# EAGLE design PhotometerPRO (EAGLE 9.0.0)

## Sheet 1 of 6: Input - Relay
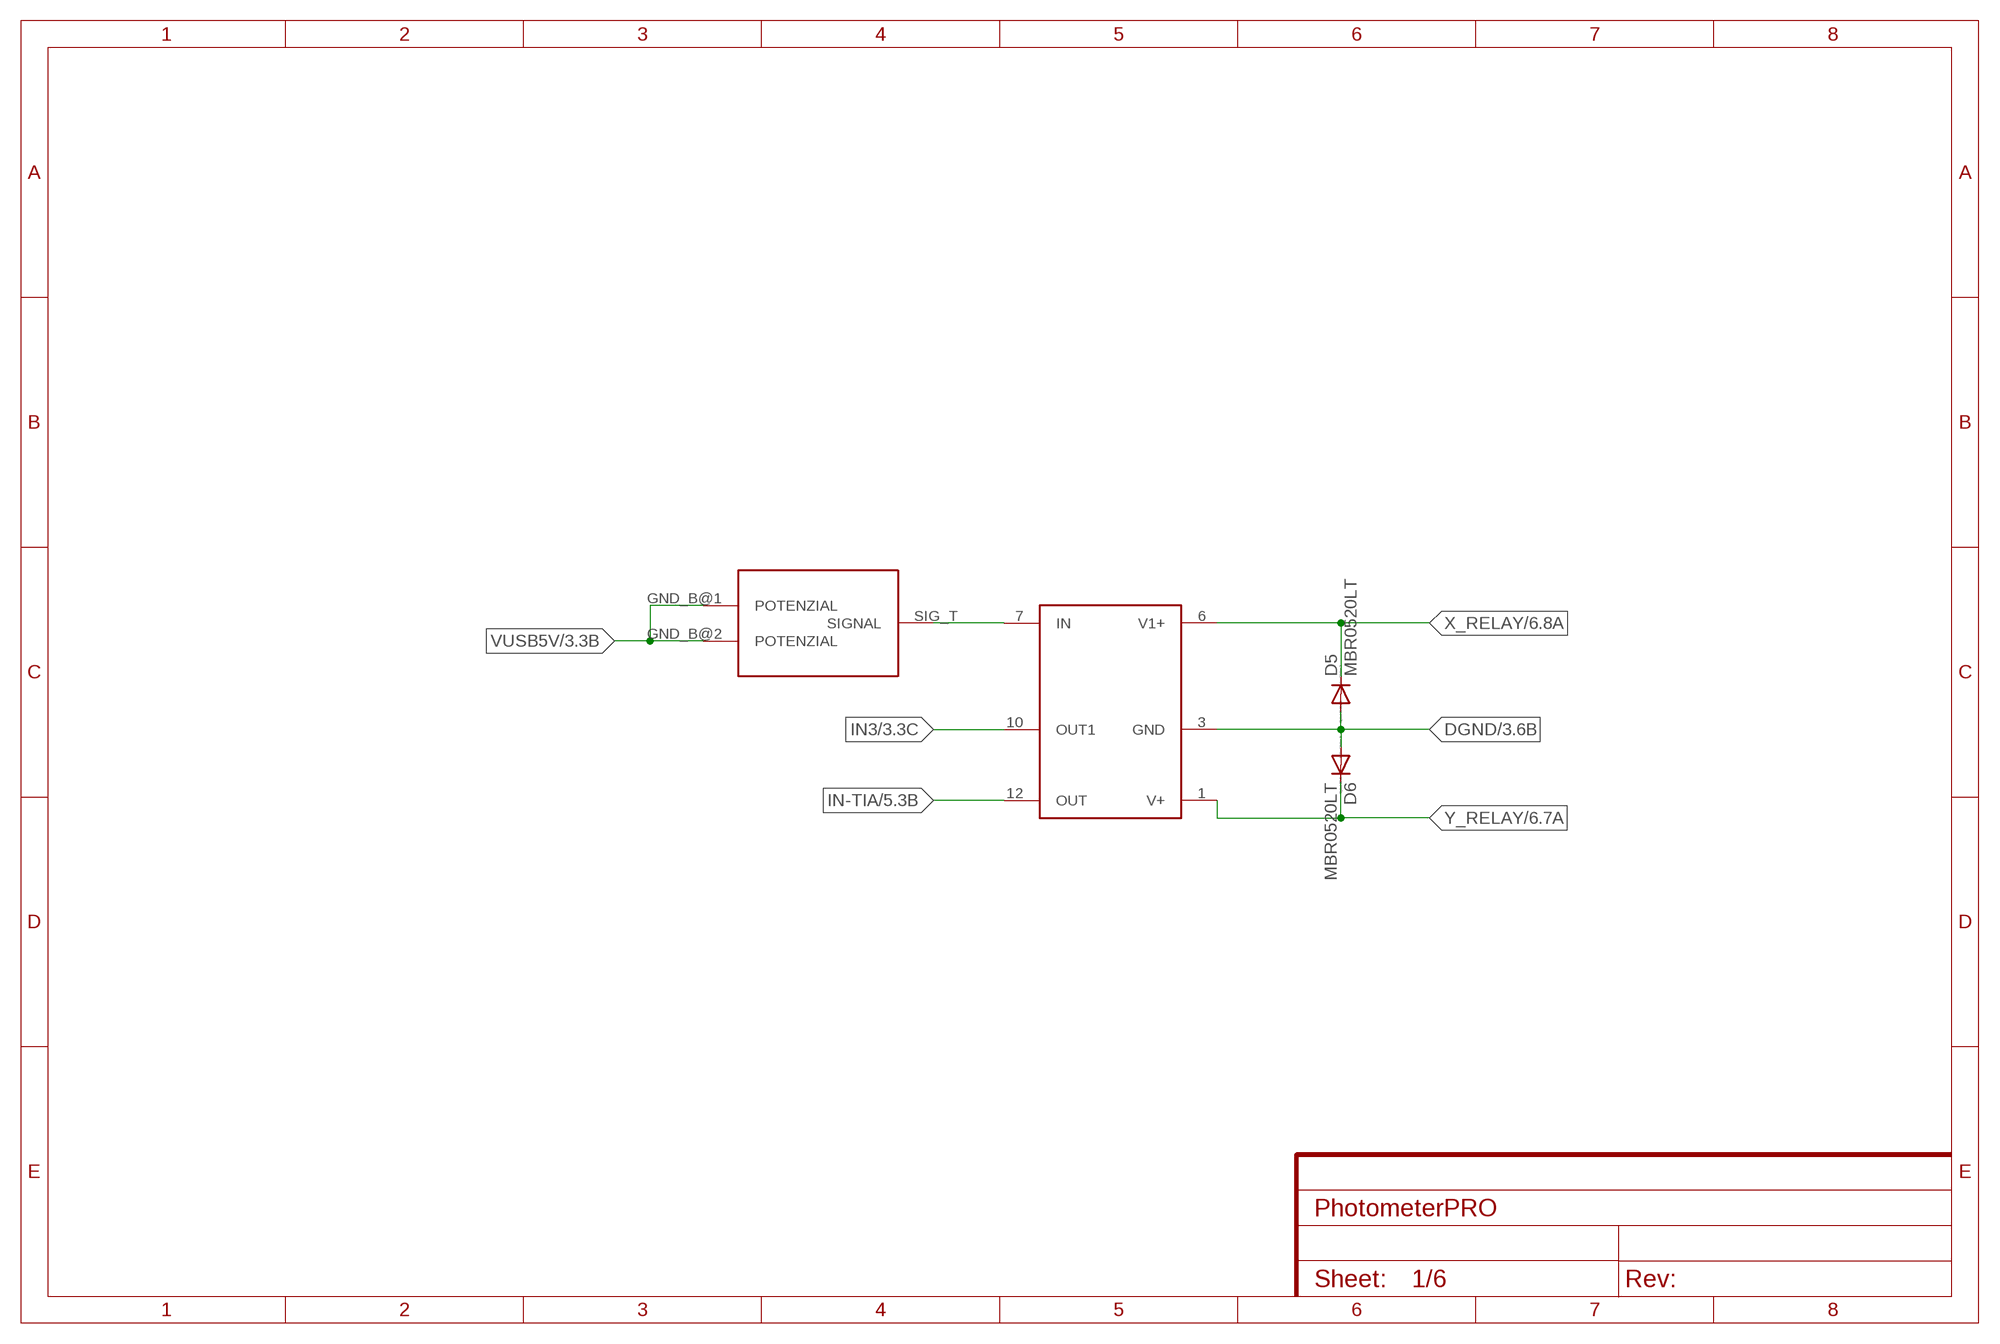
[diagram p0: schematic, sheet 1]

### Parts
CON  SMA_RAND  [SMA-RAND-PRINT]
D5  MBR0520LT  [SOD123]
D6  MBR0520LT  [SOD123]
RELAY  DS1E  [DIP12_8MM_X_13MM_DS1E]

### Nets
DGND: D5.A D6.A RELAY.3(GND) ; also sheet 3,4,6
IN3: RELAY.10(OUT1) ; also sheet 3
IN-TIA: RELAY.12(OUT) ; also sheet 5
IPD: CON.SIG_T(SIGNAL) RELAY.7(IN)
VUSB5V: CON.GND_B@1(POTENZIAL) CON.GND_B@2(POTENZIAL) ; also sheet 3,4,6
X_RELAY: D5.C RELAY.6(V1+) ; also sheet 6
Y_RELAY: D6.C RELAY.1(V+) ; also sheet 6

## Sheet 2 of 6: VFC
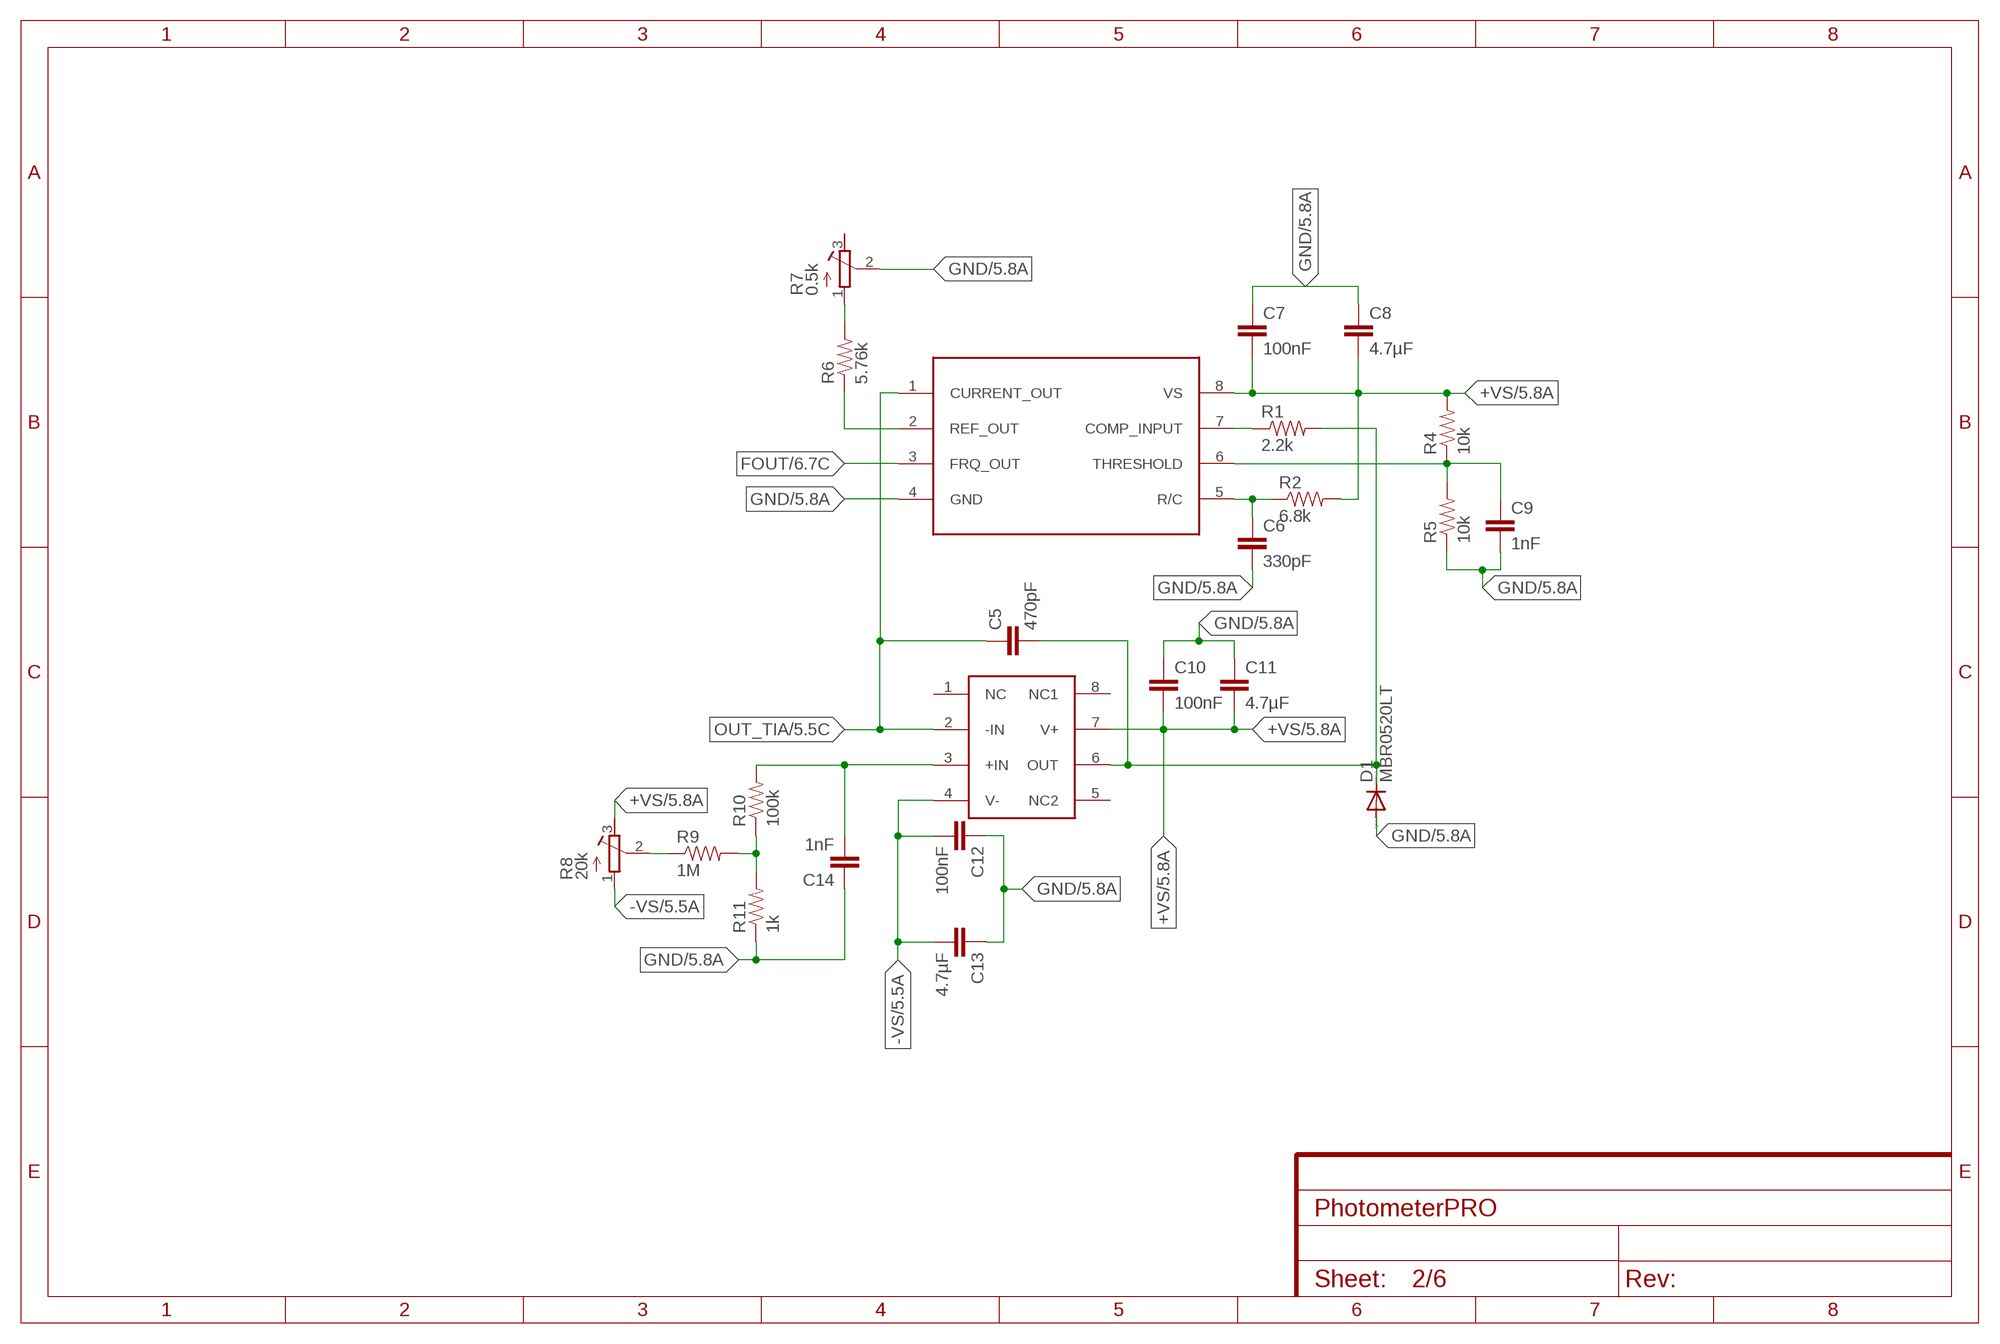
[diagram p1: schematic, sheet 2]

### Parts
C5  470pF  CAP0603-CAP  [0603-CAP]
C6  330pF  C-EUC0603K  [C0603K]
C7  100nF  C-EUC0603K  [C0603K]
C8  4.7µF  C-EUC0603K  [C0603K]
C9  1nF  C-EUC0603K  [C0603K]
C10  100nF  C-EUC0603K  [C0603K]
C11  4.7µF  C-EUC0603K  [C0603K]
C12  100nF  C-EUC0603K  [C0603K]
C13  4.7µF  C-EUC0603K  [C0603K]
C14  1nF  C-EUC0603K  [C0603K]
D1  MBR0520LT  [SOD123]
R1  2.2k  RESISTOR0603-RES  [0603-RES]
R2  6.8k  RESISTOR0805-RES  [0805]
R4  10k  RESISTOR0603-RES  [0603-RES]
R5  10k  RESISTOR0603-RES  [0603-RES]
R6  5.76k  RESISTOR0603-RES  [0603-RES]
R7  0.5k  R-TRIMMTSM53YL  [RTRIMTSM53YL]
R8  20k  R-TRIMMTS63Y  [RTRIMTS63Y]
R9  1M  RESISTOR0603-RES  [0603-RES]
R10  100k  RESISTOR0603-RES  [0603-RES]
R11  1k  RESISTOR0603-RES  [0603-RES]
U$10  OPA191  [SOIC8_4.90MMX3.91MM]
VFC  LM331  [DIP-08]

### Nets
+VS: C7.2 C8.2 C10.2 C11.2 R2.2 R4.2 R8.3(E) U$10.7(V+) VFC.8(VS) ; also sheet 5,6
-VS: C12.2 C13.2 R8.1(A) U$10.4(V-) ; also sheet 5,6
COMP_IN: R1.1 VFC.7(COMP_INPUT)
FOUT: VFC.3(FRQ_OUT) ; also sheet 6
GND: C6.2 C7.1 C8.1 C9.2 C10.1 C11.1 C12.1 C13.1 C14.1 D1.A R5.1 R7.2(S) R11.1 VFC.4(GND) ; also sheet 5,6
IN+INTE: C14.2 R10.2 U$10.3(+IN)
N$2: C5.2 D1.C R1.2 U$10.6(OUT)
N$8: C6.1 R2.1 VFC.5(R/C)
N$10: R6.1 VFC.2(REF_OUT)
N$11: C9.1 R4.1 R5.2 VFC.6(THRESHOLD)
N$12: R6.2 R7.1(A)
N$14: R9.2 R10.1 R11.2
N$15: R8.2(S) R9.1
OUT_TIA: C5.1 U$10.2(-IN) VFC.1(CURRENT_OUT) ; also sheet 5
Unconnected: R7.3(E) U$10.1(NC) U$10.5(NC2) U$10.8(NC1)

## Sheet 3 of 6: Mazet + Supply
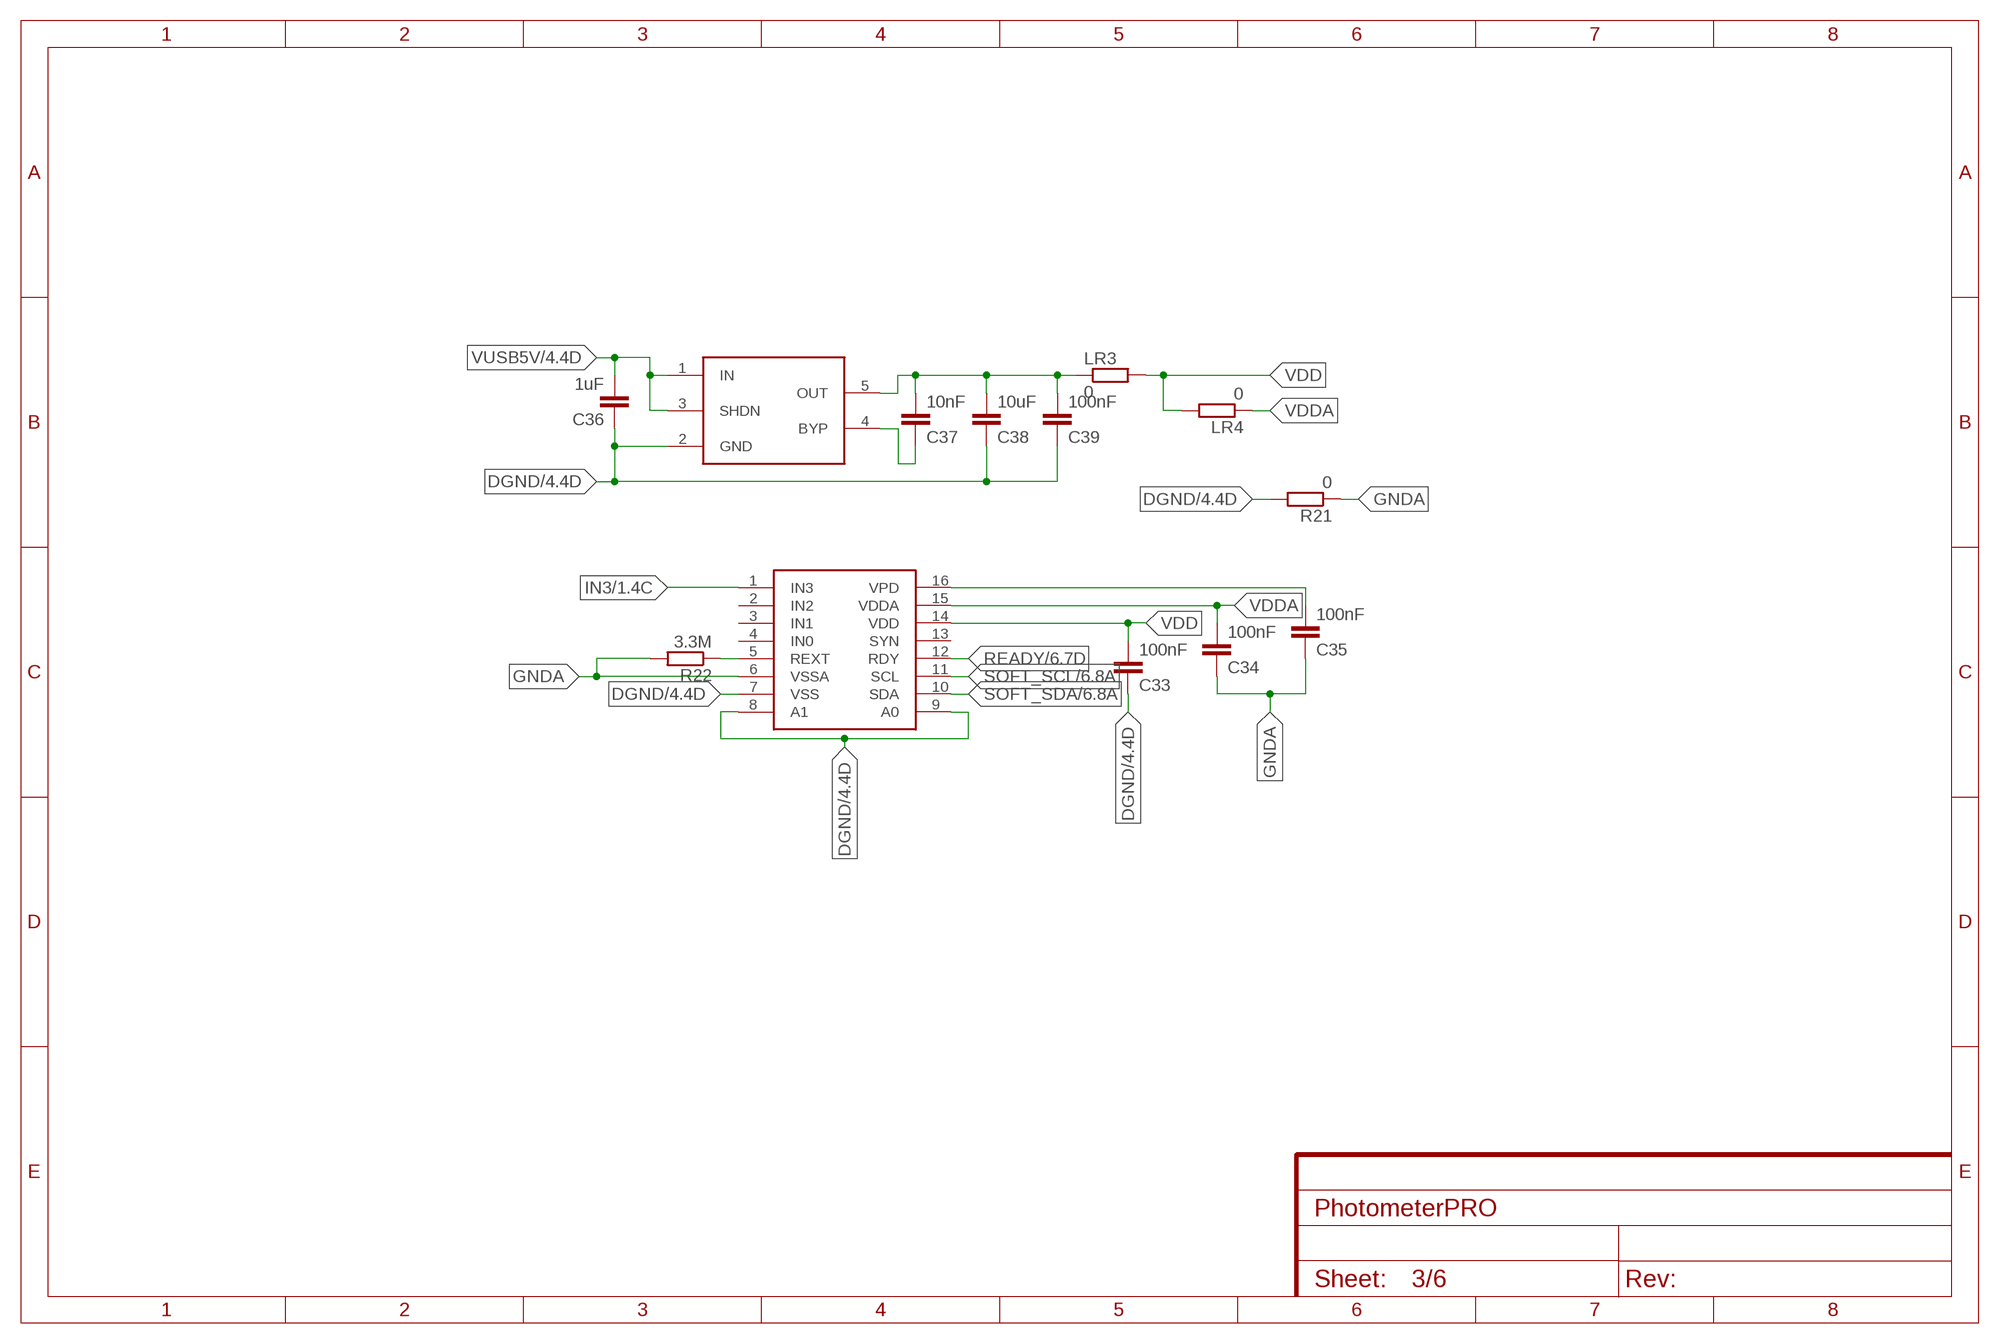
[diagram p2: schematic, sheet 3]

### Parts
C33  100nF  C-EUC0603  [C0603]
C34  100nF  C-EUC0603  [C0603]
C35  100nF  C-EUC0603  [C0603]
C36  1uF  C-EUC0603  [C0603]
C37  10nF  C-EUC0603  [C0603]
C38  10uF  C-EUC0603  [C0603]
C39  100nF  C-EUC0603  [C0603]
LDO1  LT1761  [TSOT23-5]
LR3  0  R-EU_R0603  [R0603]
LR4  0  R-EU_R0603  [R0603]
MCDC01  MCDC04  [SSOP16]
R21  0  R-EU_R0603  [R0603]
R22  3.3M  R-EU_R0603  [R0603]

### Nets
DGND: C33.1 C36.1 C38.1 C39.1 LDO1.2(GND) MCDC01.7(VSS) MCDC01.8(A1) MCDC01.9(A0) R21.2 ; also sheet 1,4,6
GNDA: C34.1 C35.1 MCDC01.6(VSSA) R21.1 R22.2
IN3: MCDC01.1(IN3) ; also sheet 1
LDO_OUT3V1: C37.2 C38.2 C39.2 LDO1.5(OUT) LR3.1
N$1: C37.1 LDO1.4(BYP)
READY: MCDC01.12(RDY) ; also sheet 6
REXT: MCDC01.5(REXT) R22.1
SOFT_SCL: MCDC01.11(SCL) ; also sheet 6
SOFT_SDA: MCDC01.10(SDA) ; also sheet 6
VDD: C33.2 LR3.2 LR4.2 MCDC01.14(VDD)
VDDA: C34.2 LR4.1 MCDC01.15(VDDA)
VPD: C35.2 MCDC01.16(VPD)
VUSB5V: C36.2 LDO1.1(IN) LDO1.3(SHDN) ; also sheet 1,4,6
Unconnected: MCDC01.2(IN2) MCDC01.3(IN1) MCDC01.4(IN0) MCDC01.13(SYN)

## Sheet 4 of 6: Display Joystik
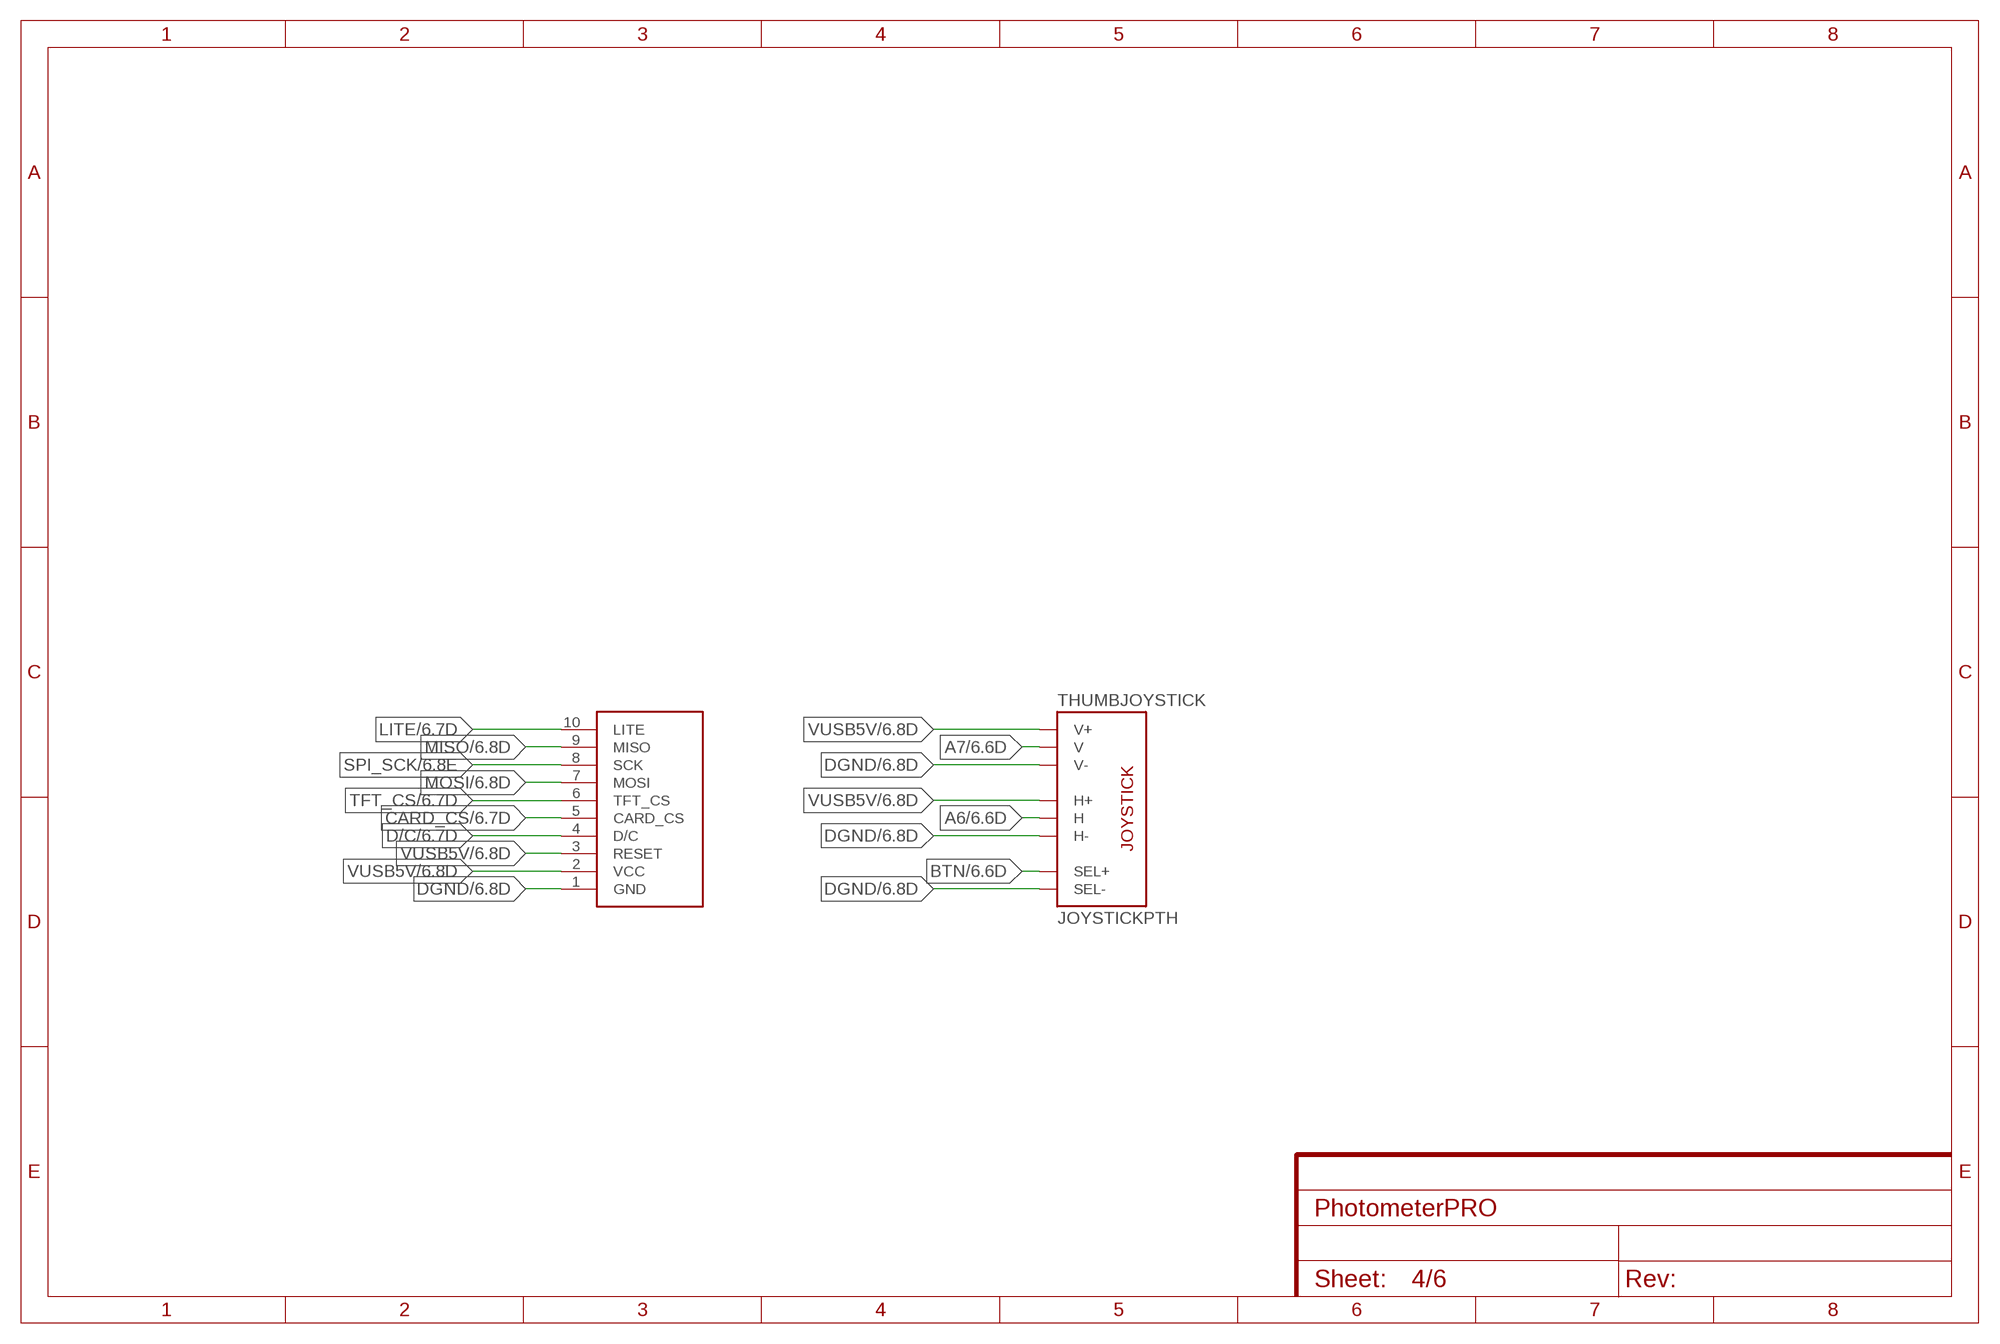
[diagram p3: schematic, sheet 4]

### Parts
DISPLAY  DISPLAY  [DISPLAY]
THUMBJOYSTICK  JOYSTICKPTH  [JOYSTICK]

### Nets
A6: THUMBJOYSTICK.H2(H) ; also sheet 6
A7: THUMBJOYSTICK.V2(V) ; also sheet 6
BTN: THUMBJOYSTICK.B1A(SEL+) ; also sheet 6
CARD_CS: DISPLAY.5(CARD_CS) ; also sheet 6
D/C: DISPLAY.4(D/C) ; also sheet 6
DGND: DISPLAY.1(GND) THUMBJOYSTICK.B2A(SEL-) THUMBJOYSTICK.H3(H-) THUMBJOYSTICK.V3(V-) ; also sheet 1,3,6
LITE: DISPLAY.10(LITE) ; also sheet 6
MISO: DISPLAY.9(MISO) ; also sheet 6
MOSI: DISPLAY.7(MOSI) ; also sheet 6
SPI_SCK: DISPLAY.8(SCK) ; also sheet 6
TFT_CS: DISPLAY.6(TFT_CS) ; also sheet 6
VUSB5V: DISPLAY.2(VCC) DISPLAY.3(RESET) THUMBJOYSTICK.H1(H+) THUMBJOYSTICK.V1(V+) ; also sheet 1,3,6

## Sheet 5 of 6: TIA
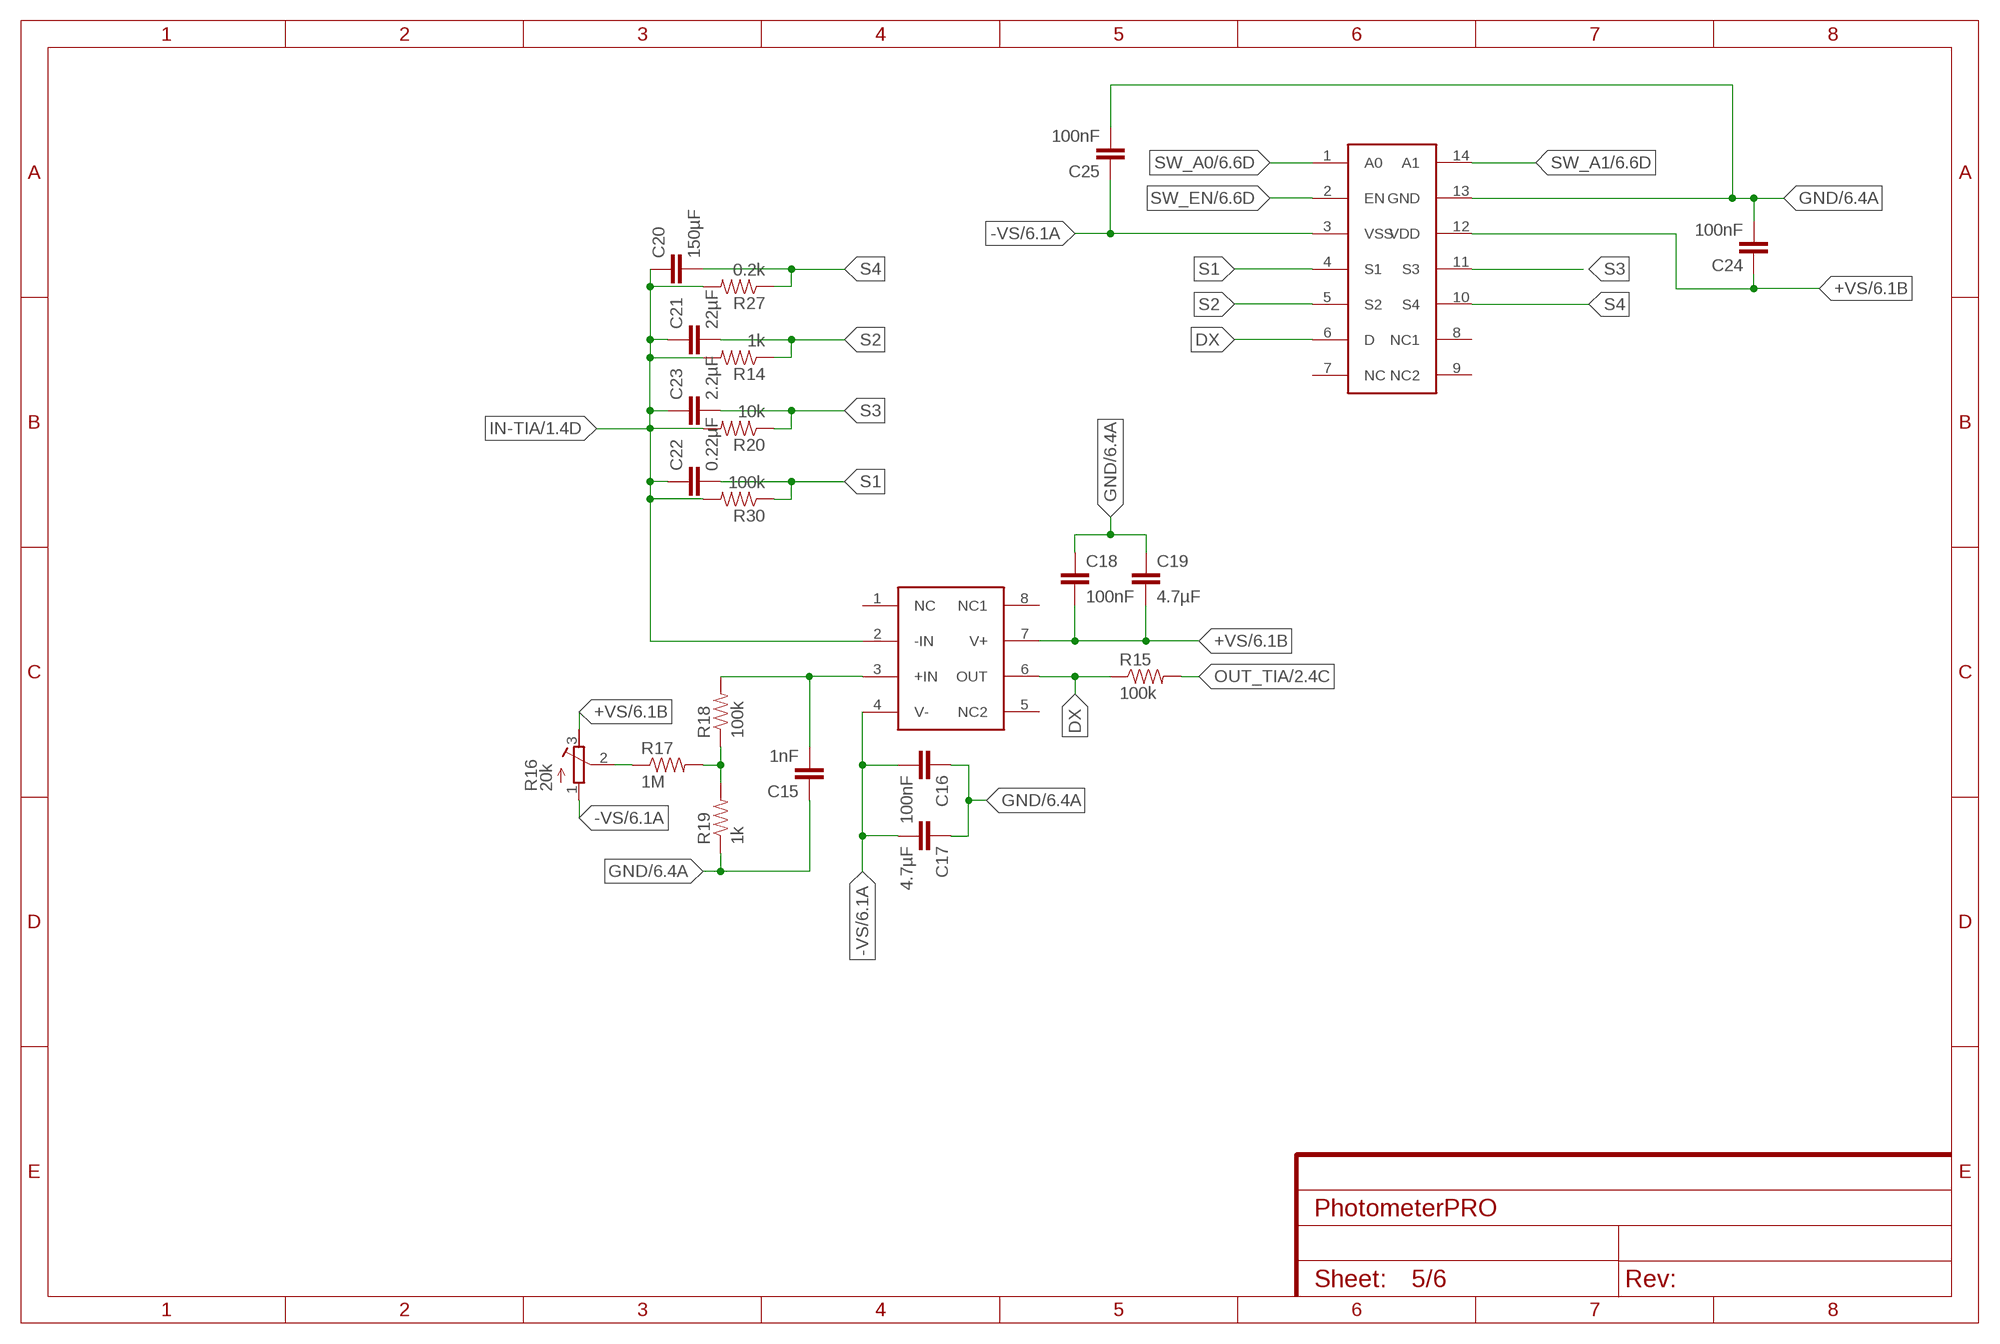
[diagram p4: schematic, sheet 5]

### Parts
C15  1nF  C-EUC0603K  [C0603K]
C16  100nF  C-EUC0603K  [C0603K]
C17  4.7µF  C-EUC0603K  [C0603K]
C18  100nF  C-EUC0603K  [C0603K]
C19  4.7µF  C-EUC0603K  [C0603K]
C20  150µF  C-EUC1206  [C1206]
C21  22µF  C-EUC0805  [C0805]
C22  0.22µF  C-EUC0603  [C0603]
C23  2.2µF  C-EUC0805  [C0805]
C24  100nF  C-EUC0603K  [C0603K]
C25  100nF  C-EUC0603K  [C0603K]
R14  1k  RESISTOR0603-RES  [0603-RES]
R15  100k  RESISTOR0603-RES  [0603-RES]
R16  20k  R-TRIMMTS63Y  [RTRIMTS63Y]
R17  1M  RESISTOR0603-RES  [0603-RES]
R18  100k  RESISTOR0603-RES  [0603-RES]
R19  1k  RESISTOR0603-RES  [0603-RES]
R20  10k  RESISTOR0603-RES  [0603-RES]
R27  0.2k  RESISTOR1206  [1206]
R30  100k  RESISTOR0603-RES  [0603-RES]
U$1  ADG1404  [TSSOP14-0.65-5X4.4MM]
U$12  OPA191  [SOIC8_4.90MMX3.91MM]

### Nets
+VS: C18.2 C19.2 C24.1 R16.3(E) U$1.12(VDD) U$12.7(V+) ; also sheet 2,6
-VS: C16.2 C17.2 C25.1 R16.1(A) U$1.3(VSS) U$12.4(V-) ; also sheet 2,6
DX: R15.1 U$1.6(D) U$12.6(OUT)
GND: C15.1 C16.1 C17.1 C18.1 C19.1 C24.2 C25.2 R19.1 U$1.13(GND) ; also sheet 2,6
IN+TIA: C15.2 R18.2 U$12.3(+IN)
IN-TIA: C20.1 C21.1 C22.1 C23.1 R14.2 R20.2 R27.2 R30.2 U$12.2(-IN) ; also sheet 1
N$21: R17.2 R18.1 R19.2
N$22: R16.2(S) R17.1
OUT_TIA: R15.2 ; also sheet 2
S1: C22.2 R30.1 U$1.4(S1)
S2: C21.2 R14.1 U$1.5(S2)
S3: C23.2 R20.1 U$1.11(S3)
S4: C20.2 R27.1 U$1.10(S4)
SW_A0: U$1.1(A0) ; also sheet 6
SW_A1: U$1.14(A1) ; also sheet 6
SW_EN: U$1.2(EN) ; also sheet 6
Unconnected: U$1.7(NC) U$1.8(NC1) U$1.9(NC2) U$12.1(NC) U$12.5(NC2) U$12.8(NC1)

## Sheet 6 of 6: µC-Nano Versorgung
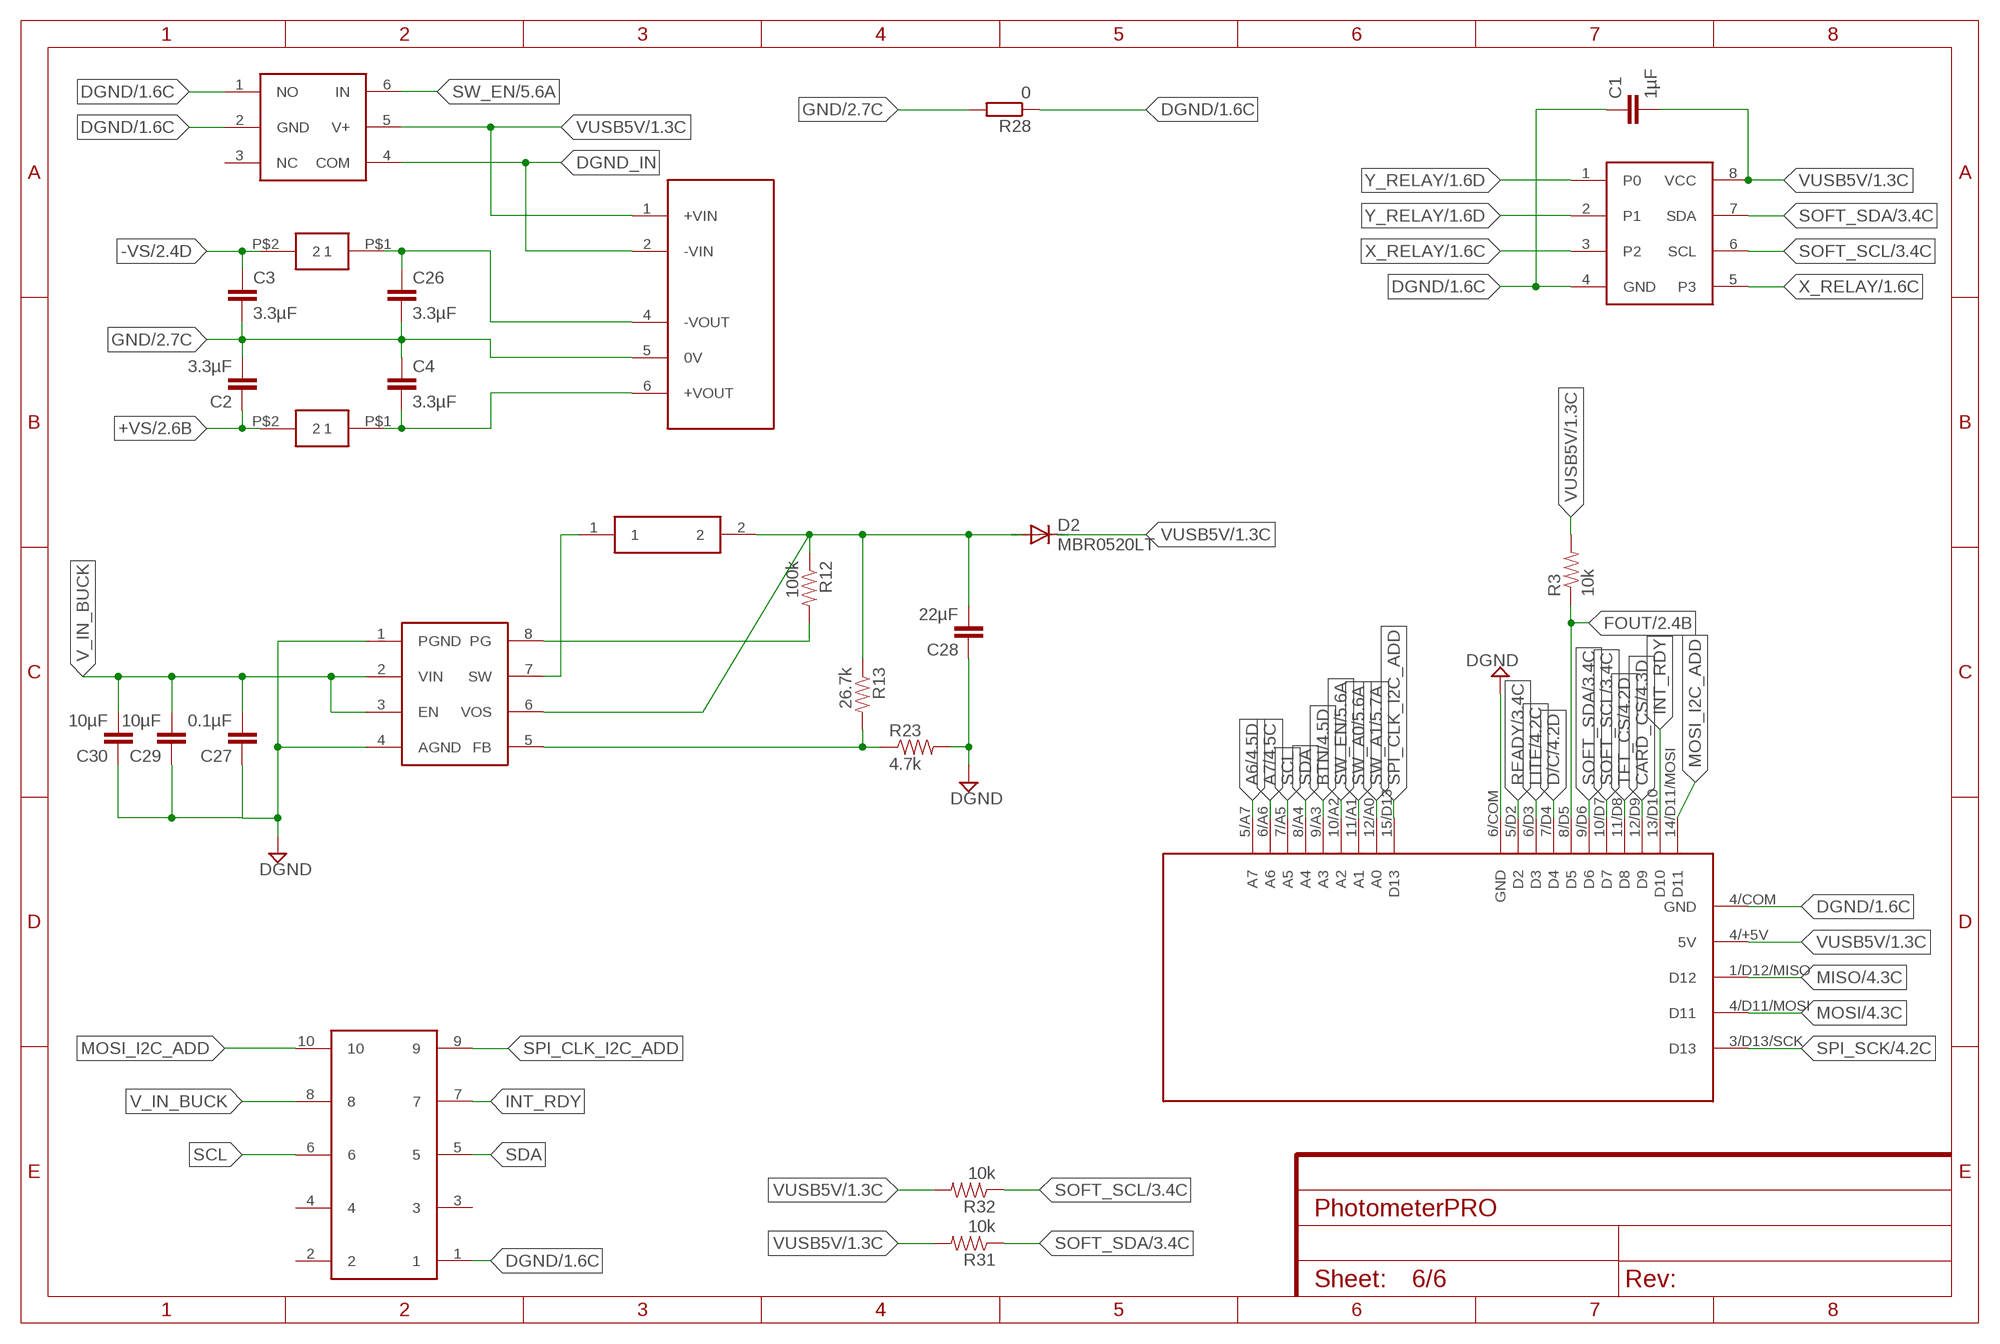
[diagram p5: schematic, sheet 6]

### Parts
C1  1µF  C-EUC0603K  [C0603K]
C2  3.3µF  C-EUC0603K  [C0603K]
C3  3.3µF  C-EUC0603K  [C0603K]
C4  3.3µF  C-EUC0603K  [C0603K]
C26  3.3µF  C-EUC0603K  [C0603K]
C27  0.1µF  C-EUC0603K  [C0603K]
C28  22µF  C-EUC0603K  [C0603K]
C29  10µF  C-EUC0603K  [C0603K]
C30  10µF  C-EUC0603K  [C0603K]
D2  MBR0520LT  [SOD123]
R3  10k  RESISTOR0603-RES  [0603-RES]
R12  100k  RESISTOR0603-RES  [0603-RES]
R13  26.7k  RESISTOR0603-RES  [0603-RES]
R23  4.7k  RESISTOR0603-RES  [0603-RES]
R28  0  R-EU_R0603  [R0603]
R31  10k  RESISTOR0603-RES  [0603-RES]
R32  10k  RESISTOR0603-RES  [0603-RES]
U$2  KMP_100µH  KMP  [KMP]
U$3  HEADER_10POL  [BOX_HEADER_2.54MM]
U$4  KMP_100µH  KMP  [KMP]
U$6  TS5A3159A  [SOT23-6]
U$7  0  PCA9536  [SOIC8_4.90MMX3.91MM]
U$9  LPS3015  [LPS3015]
U$11  NMA0515SC  [SIP7]
U$13  NANO_V2  [NANO_V2]
U$14  TPS62160  [POWER-SOP8]

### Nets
5.5VBUCK: C28.2 D2.A R12.1 R13.1 U$9.2 U$14.6(VOS)
+VS: C2.1 U$4.P$2 ; also sheet 2,5
-VS: C3.1 U$2.P$2 ; also sheet 2,5
A6: U$13.5/A7(A7) ; also sheet 4
A7: U$13.6/A6(A6) ; also sheet 4
BTN: U$13.9/A3(A3) ; also sheet 4
CARD_CS: U$13.12/D9(D9) ; also sheet 4
D/C: U$13.7/D4(D4) ; also sheet 4
DGND: C1.1 C27.1 C28.1 C29.1 C30.1 R23.2 R28.1 U$3.1 U$6.1(NO) U$6.2(GND) U$7.4(GND) U$13.4/COM(GND) U$13.6/COM(GND) U$14.1(PGND) U$14.4(AGND) ; also sheet 1,3,4
DGND_IN: U$6.4(COM) U$11.2(-VIN)
FOUT: R3.1 U$13.8/D5(D5) ; also sheet 2
GND: C2.2 C3.2 C4.1 C26.2 R28.2 U$11.5(0V) ; also sheet 2,5
INT_RDY: U$3.7 U$13.13/D10(D10)
LITE: U$13.6/D3(D3) ; also sheet 4
MISO: U$13.1/D12/MISO(D12) ; also sheet 4
MOSI: U$13.4/D11/MOSI(D11) ; also sheet 4
MOSI_I2C_ADD: U$3.10 U$13.14/D11/MOSI(D11)
N$4: C4.2 U$4.P$1 U$11.6(+VOUT)
N$6: C26.1 U$2.P$1 U$11.4(-VOUT)
N$7: R13.2 R23.1 U$14.5(FB)
N$17: R12.2 U$14.8(PG)
N$18: U$9.1 U$14.7(SW)
READY: U$13.5/D2(D2) ; also sheet 3
SCL: U$3.6 U$13.7/A5(A5)
SDA: U$3.5 U$13.8/A4(A4)
SOFT_SCL: R32.1 U$7.6(SCL) U$13.10/D7(D7) ; also sheet 3
SOFT_SDA: R31.1 U$7.7(SDA) U$13.9/D6(D6) ; also sheet 3
SPI_CLK_I2C_ADD: U$3.9 U$13.15/D13(D13)
SPI_SCK: U$13.3/D13/SCK(D13) ; also sheet 4
SW_A0: U$13.11/A1(A1) ; also sheet 5
SW_A1: U$13.12/A0(A0) ; also sheet 5
SW_EN: U$6.6(IN) U$13.10/A2(A2) ; also sheet 5
TFT_CS: U$13.11/D8(D8) ; also sheet 4
V_IN_BUCK: C27.2 C29.2 C30.2 U$3.8 U$14.2(VIN) U$14.3(EN)
VUSB5V: C1.2 D2.C R3.2 R31.2 R32.2 U$6.5(V+) U$7.8(VCC) U$11.1(+VIN) U$13.4/+5V(5V) ; also sheet 1,3,4
X_RELAY: U$7.3(P2) U$7.5(P3) ; also sheet 1
Y_RELAY: U$7.1(P0) U$7.2(P1) ; also sheet 1
Unconnected: U$3.2 U$3.3 U$3.4 U$6.3(NC)

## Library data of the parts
C1-C4 C6-C30 C33-C39 = rcl:C-EU: CAPACITOR, European symbol
C5 = SparkFun-Passives:CAP: Capacitor
CON = VFC_lib:SMA_RAND
D1 D2 D5 D6 = VFC_lib:MBR0520LT: SCHOTTKY BARRIER RECTIFIER
DISPLAY = Lego:DISPLAY
LDO1 = OpenPhotonicsLib:LT1761
LR3 LR4 R21 R22 = rcl:R-EU_: RESISTOR, European symbol
MCDC01 = BachelorLib:MCDC04
R1-R6 R9-R15 R17-R20 R23 R27 R30-R32 = SparkFun-Passives:RESISTOR: Resistor
R7 R8 R16 = resistor:R-TRIMM: Trimm resistor
R28 = resistor:R-EU_: RESISTOR, European symbol
RELAY = VFC_lib:DS1E
THUMBJOYSTICK = SparkFun-Electromechanical:JOYSTICK: Thumb Joystick Joystick commonly found in PS2 controllers. Two pots and a select switch. Footprint proven. Spark Fun Electronics SKU : COM-09032
U$1 = VFC_lib:ADG1404
U$2 U$4 = VFC_lib:KMP
U$3 = VFC_lib:HEADER_10POL
U$6 = VFC_lib:TS5A3159A
U$7 = VFC_lib:PCA9536
U$9 = VFC_lib:LPS3015
U$10 U$12 = VFC_lib:OPA191
U$11 = VFC_lib:NMA0515SC
U$13 = VFC_lib:NANO_V2
U$14 = VFC_lib:TPS62160
VFC = VFC_lib:LM331

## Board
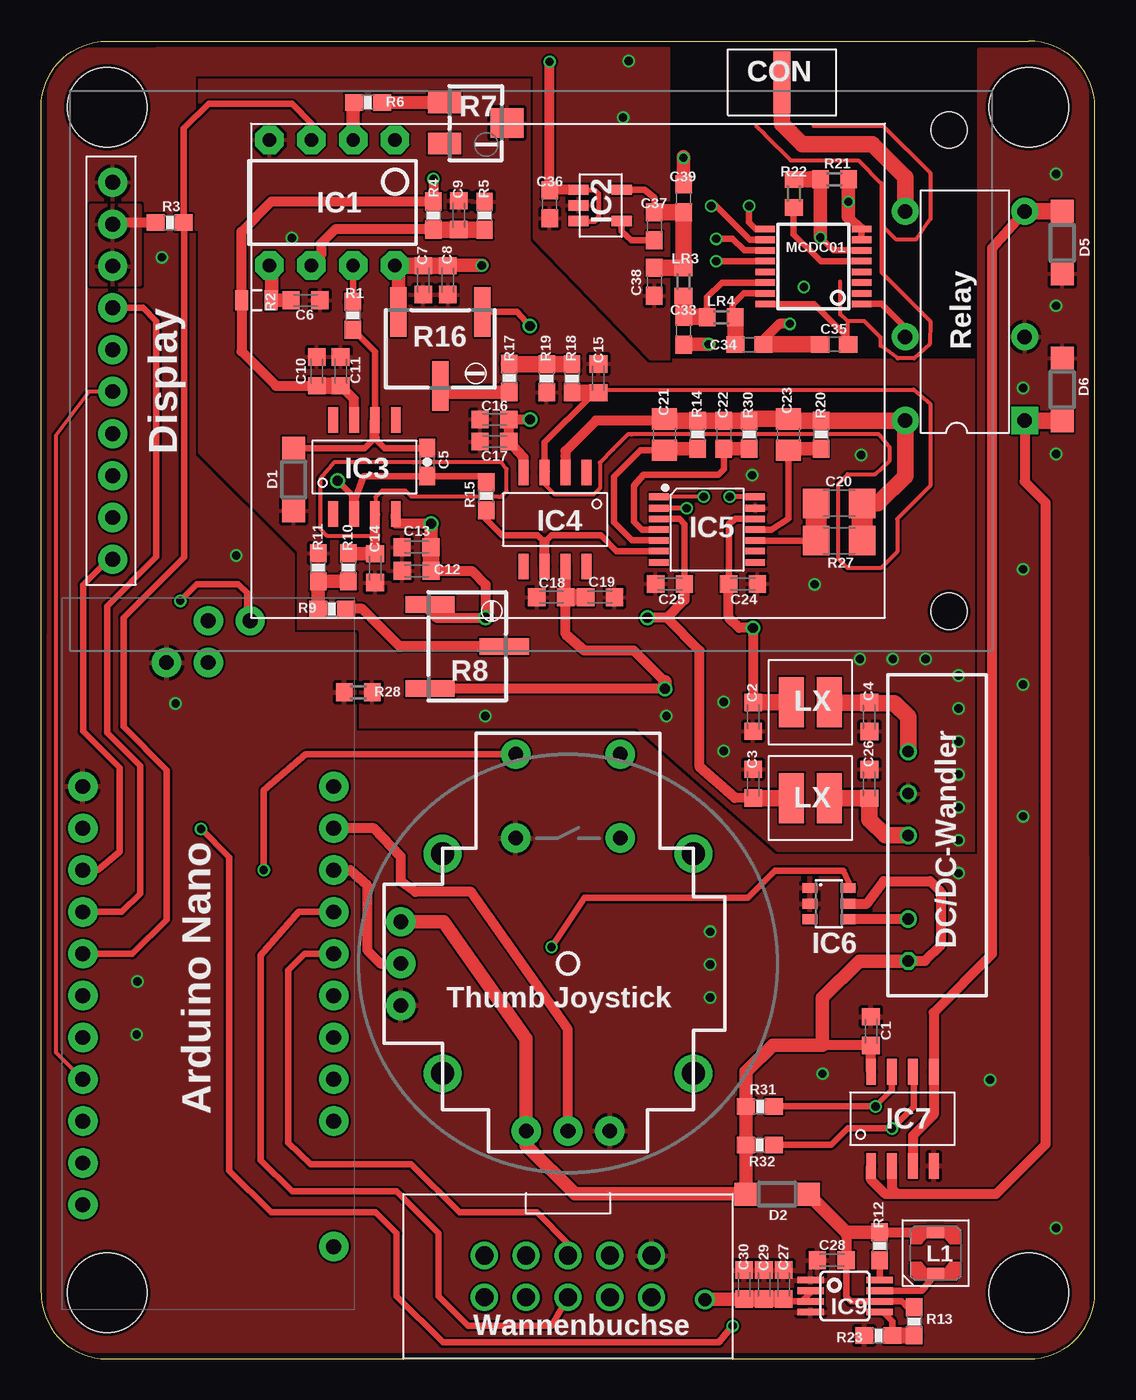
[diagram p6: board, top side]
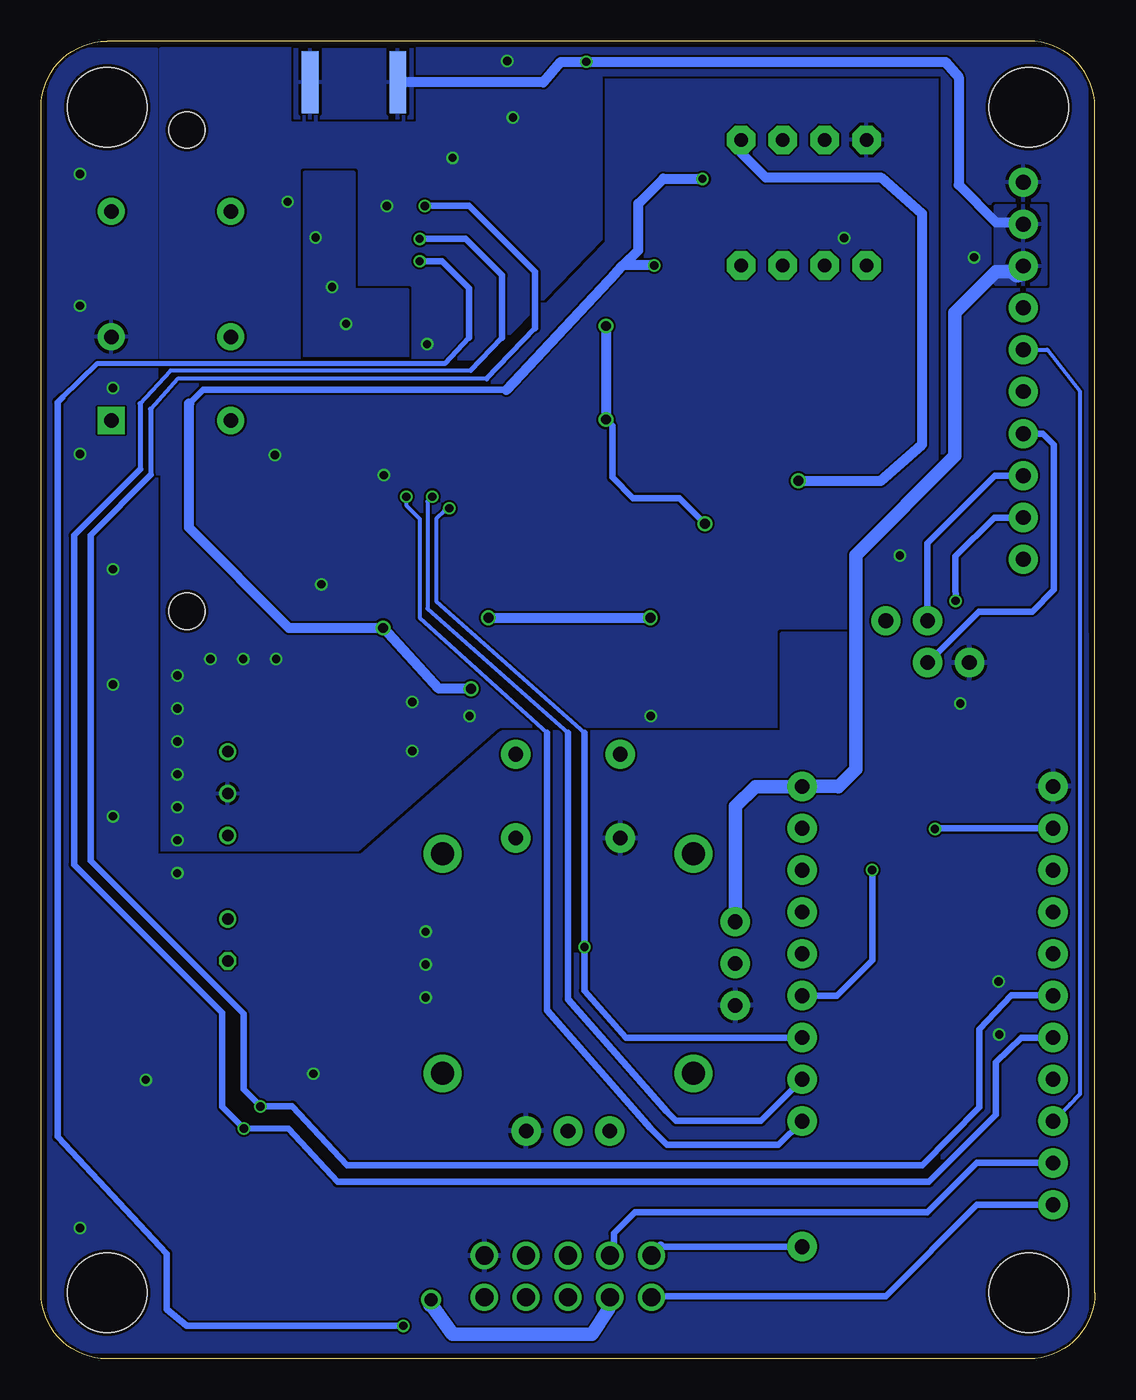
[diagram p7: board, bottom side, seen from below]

Size 64 x 80 mm. Coordinates in mm from the lower left corner, seen from the top.
Outline: 0,4 arc90 4,0 60,0 arc90 64,4 64,76 arc90 60,80 4,80 arc90 0,76 0,4
Copper layers (1*16): Top 0.018mm / dielectric 1.55mm / Bottom 0.018mm
Design rules "Multi-CB_2L_125um-Tracks_OL35um": minimum track width 0.125mm, minimum drill 0.2mm, track to track 0.125mm, track to pad 0.125mm, pad to pad 0.125mm, via to via 0.125mm, smd to smd 0mil, copper to edge 0.2mm, drill to drill 0.2mm, minimum pad ring 0.125mm, minimum via ring 0.125mm, stop-mask expansion 2mil, vias tented up to drill 0.45mm, thermal gap 0.2mm
Holes 4.82 mm at 4,76 60,76 60,4 4,4

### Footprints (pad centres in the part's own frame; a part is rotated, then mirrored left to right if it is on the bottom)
C0603K = smd 1.05 x 1.08: 1 -0.875,0; 2 0.875,0
0603-CAP = smd 1.1 x 1: 1 -0.85,0; 2 0.85,0
C1206 = smd 1.6 x 1.8: 1 -1.4,0; 2 1.4,0
C0805 = smd 1.3 x 1.5: 1 -0.95,0; 2 0.95,0
C0603 = smd 1.1 x 1: 1 -0.85,0; 2 0.85,0
SMA-RAND-PRINT = smd 3.75 x 1.02 bottom: GND_B@1 0,2.665; GND_B@2 0,-2.665 | smd 3.75 x 1.02: SIG_T 0,0
SOD123 = smd 1.4 x 1.4: A 1.9,0; C -1.9,0
DISPLAY = drill 0.9 pad 1.778: 1 -25.4,11.43; 2 -25.4,8.89; 3 -25.4,6.35; 4 -25.4,3.81; 5 -25.4,1.27; 6 -25.4,-1.27; 7 -25.4,-3.84; 8 -25.4,-6.38; 9 -25.4,-8.92; 10 -25.4,-11.46 | hole 2.2: 25.4,-14.605; 25.4,14.605
TSOT23-5 = smd 0.62 x 1.22: 1 0,-2.62; 2 0.95,-2.62; 3 1.9,-2.62; 4 1.9,0; 5 0,0
R0603 = smd 1 x 1.1: 1 -0.85,0; 2 0.85,0
SSOP16 = smd 0.4 x 1.2: 1 -2.275,-2.925; 2 -1.625,-2.925; 3 -0.975,-2.925; 4 -0.325,-2.925; 5 0.325,-2.925; 6 0.975,-2.925; 7 1.625,-2.925; 8 2.275,-2.925; 9 2.275,2.925; 10 1.625,2.925; 11 0.975,2.925; 12 0.325,2.925; 13 -0.325,2.925; 14 -0.975,2.925; 15 -1.625,2.925; 16 -2.275,2.925
0603-RES = smd 1.1 x 1: 1 -0.85,0; 2 0.85,0
0805 = smd 0.8 x 1.2: 1 -0.9,0; 2 0.9,0
RTRIMTSM53YL = smd 1.3 x 2: 1 -1.25,-1.9; 3 1.25,-1.9 | smd 1.8 x 2: 2 0,1.9
RTRIMTS63Y = smd 1 x 3: 1 -2.55,-2.25; 2 0,2.25; 3 2.55,-2.25
1206 = smd 1.6 x 1.8: 1 -1.4,0; 2 1.4,0
DIP12_8MM_X_13MM_DS1E = drill 0.889 pad 1.651 square: 1 -7.62,-4.128 | drill 0.889 pad 1.651: 3 -2.54,-4.128; 6 5.08,-4.128; 7 5.08,3.127; 10 -2.54,3.127; 12 -7.62,3.127
JOYSTICK = drill 0.9 pad 1.778: B1A -3.175,12.7; B1B 3.175,12.7; B2A -3.175,7.62; B2B 3.175,7.62 | drill 0.889 pad 1.778: H1 -2.54,-10.16; H2 0,-10.16; H3 2.54,-10.16; V1 -10.16,2.54; V2 -10.16,0; V3 -10.16,-2.54 | drill 1.397 pad 2.286: MOUNT1 -7.62,6.668; MOUNT2 -7.62,-6.668; MOUNT3 7.62,-6.668; MOUNT4 7.62,6.668
TSSOP14-0.65-5X4.4MM = smd 0.4 x 1.2: 1 -2,-2.925; 2 -1.3,-2.925; 3 -0.65,-2.925; 4 0,-2.925; 5 0.65,-2.925; 6 1.3,-2.925; 7 2,-2.925; 8 2,2.925; 9 1.3,2.925; 10 0.65,2.925; 11 0,2.925; 12 -0.65,2.925; 13 -1.3,2.925; 14 -2,2.925
KMP = smd 1.52 x 3.05: P$1 -1.145,0; P$2 1.145,0
BOX_HEADER_2.54MM = drill 1.1: 1 -1.27,5.08; 2 1.27,5.08; 3 -1.27,2.54; 4 1.27,2.54; 5 -1.27,0; 6 1.27,0; 7 -1.27,-2.54; 8 1.27,-2.54; 9 -1.27,-5.08; 10 1.27,-5.08
SOT23-6 = smd 0.6 x 0.9: 1 -0.95,-1.15; 2 0,-1.15; 3 0.95,-1.15; 4 0.95,1.15; 5 0,1.15; 6 -0.95,1.15
SOIC8_4.90MMX3.91MM = smd 0.6 x 1.55: 1 -1.27,-5.715; 2 0,-5.715; 3 1.27,-5.715; 4 2.54,-5.715; 5 2.54,0; 6 1.27,0; 7 0,0; 8 -1.27,0
LPS3015 = smd 0.76 x 1.02: 1 -1.27,0; 2 1.27,0.01
SIP7 = drill 0.7 pad 1.016 octagon: 1 -7.62,1.75 | drill 0.7 pad 1.016: 2 -5.08,1.75; 4 0,1.75; 5 2.54,1.75; 6 5.08,1.75
NANO_V2 = drill 0.9 pad 1.778: 1/D12/MISO 41.808,6.35; 3/D13/SCK 41.808,8.89; 4/+5V 31.75,1.27; 4/COM 31.75,16.51; 4/D11/MOSI 39.268,8.89; 5/A7 29.21,1.27; 5/D2 29.21,16.51; 6/A6 26.67,1.27; 6/COM 39.268,11.43; 6/D3 26.67,16.51; 7/A5 24.13,1.27; 7/D4 24.13,16.51; 8/A4 21.59,1.27; 8/D5 21.59,16.51; 9/A3 19.05,1.27; 9/D6 19.05,16.51; 10/A2 16.51,1.27; 10/D7 16.51,16.51; 11/A1 13.97,1.27; 11/D8 13.97,16.51; 12/A0 11.43,1.27; 12/D9 11.43,16.51; 13/D10 8.89,16.51; 14/D11/MOSI 6.35,16.51; 15/D13 3.81,1.27
POWER-SOP8 = smd 0.4 x 1.6: 1 -0.975,-2.1; 2 -0.325,-2.1; 3 0.325,-2.1; 4 0.975,-2.1; 5 0.975,2.1; 6 0.325,2.1; 7 -0.325,2.1; 8 -0.975,2.1
DIP-08 = drill 0.813 pad 1.727 octagon: 1 -3.81,-3.81; 2 -1.27,-3.81; 3 1.27,-3.81; 4 3.81,-3.81; 5 3.81,3.81; 6 1.27,3.81; 7 -1.27,3.81; 8 -3.81,3.81

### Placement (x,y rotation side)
C1  50.41,19.9 270 top
C2  43.24,38.98 270 top
C3  43.24,34.92 90 top
C4  50.3,38.97 90 top
C5  23.44,54.45 90 top
C6  16.05,64.26 0 top
C7  23.21,65.49 90 top
C8  24.7,65.49 90 top
C9  25.37,69.43 90 top
C10  16.74,59.95 270 top
C11  18.19,59.95 270 top
C12  22.81,47.84 0 top
C13  22.8,49.28 0 top
C14  20.29,48.01 90 top
C15  33.85,59.53 270 top
C16  27.53,57.03 0 top
C17  27.53,55.69 0 top
C18  30.98,46.24 0 top
C19  33.95,46.25 180 top
C20  48.47,51.94 180 top
C21  37.86,56.11 270 top
C22  41.47,56.11 270 top
C23  45.38,56.11 270 top
C24  42.63,47.04 0 top
C25  38.2,47.04 180 top
C26  50.3,34.91 90 top
C27  45.09,4.52 270 top
C28  48.03,5.98 0 top
C29  43.9,4.51 270 top
C30  42.7,4.51 270 top
C33  39.01,62.41 90 top
C34  43.02,61.58 180 top
C35  48.17,61.58 0 top
C36  30.88,70.11 90 top
C37  37.25,68.76 90 top
C38  37.25,65.39 90 top
C39  39.01,70.46 270 top
CON  45,77.5 90 top
D1  15.34,53.39 270 top
D2  44.71,10 0 top
D5  62.01,67.77 270 top
D6  62.01,58.85 90 top
DISPLAY  29.75,60 0 top
LDO1  35.26,70.98 270 top
LR3  39.01,65.39 270 top
LR4  41.31,63.24 180 top
MCDC01  46.91,66.32 90 top
R1  18.94,63.34 270 top
R2  13.08,64.26 180 top
R3  7.81,68.99 180 top
R4  23.83,69.42 90 top
R5  26.93,69.41 270 top
R6  19.85,76.28 0 top
R7  26.39,75.03 270 top
R8  25.87,43.26 270 top
R9  17.66,45.53 180 top
R10  18.67,48.06 90 top
R11  16.82,48.05 270 top
R12  50.93,6.85 270 top
R13  53.02,2.27 270 top
R14  39.87,56.11 90 top
R15  27.03,52.38 90 top
R16  24.25,61.31 180 top
R17  28.45,59.55 90 top
R18  32.24,59.53 270 top
R19  30.7,59.53 90 top
R20  47.37,56.11 90 top
R21  48.18,71.62 0 top
R22  45.72,70.75 90 top
R23  50.86,1.4 180 top
R27  48.47,49.68 0 top
R28  19.26,40.47 0 top
R30  43.02,56.11 90 top
R31  43.66,15.32 180 top
R32  43.65,12.98 180 top
RELAY  55.61,64.59 90 top
THUMBJOYSTICK  32,24 0 top
U$1  40.45,50.34 270 top
U$2  46.72,34.04 180 top
U$3  32,5 270 top
U$4  46.72,39.86 180 top
U$6  47.85,27.64 270 top
U$7  51.68,17.43 0 top
U$9  54.33,6.42 90 top
U$10  19,57 0 top
U$11  54.42,31.78 90 top
U$12  31.85,48.1 180 top
U$13  19.04,3 90 top
U$14  48.83,3.81 270 top
VFC  17.68,70.2 180 top

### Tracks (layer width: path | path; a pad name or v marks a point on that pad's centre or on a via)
5.5VBUCK
  Top 0.406: C28.2 48.9,3.76 49.17,3.48 U$14.6 52.27,3.48 52.64,3.11 R13.1
  Top 0.61: R12.1 52.97,7.7 U$9.2 | 49.06,7.7 48.9,7.49 C28.2
  Top 0.813: R12.1 49.06,7.7 48.92,7.7 D2.A | C28.2
  Top 1.016: 46.64,9.98 D2.A
+VS  (via drill 0.5, 0.6)
  Top 0.406: U$1.12 42.16,50.99 41.77,50.7 41.77,47.05 C24.1
  Top 0.61: U$4.P$2 45.58,40.31 | U$4.P$2 | U$4.P$2 | C24.1 41.76,45.03 42.41,44.38 v43.23,44.38 43.23,39.87 | v37.89,40.69 22.64,40.69 R8.3 | 14,70.27 12.18,68.43 R2.2 12.18,61.17 14.27,59.08 C10.2 16.75,59.06 | U$12.7 31.85,46.25 C18.2 | U$10.7 19,58.27 C11.2 | 37.89,41.11 36,43 33,43 31.85,44 31.85,46.1 C18.2 | C18.2 | v23.83,71.64 R4.2 23.85,70.27 23.85,70.28 14,70.28 14,70.27 | 14,70.27
  Top 0.813: 43.23,39.87 C2.1 | 24.69,66.36 C8.2 | C8.2 | v37.89,40.69 37.89,41.11 | v26.77,66.38 24.72,66.38 C8.2 | R16.3 21.71,66.17 VFC.8 | C10.2
  Top 1.016: C2.1 U$4.P$2 | C10.2 C11.2 | C19.2 C18.2 | 24.69,66.36 23.23,66.36 C7.2 21.51,66.37 VFC.8
  Bottom 0.406: 35.74,58.83 54.17,58.83 55,58
  Bottom 0.61: 35.74,58.83 29.1,65.94 | 29.1,65.94 29,66.04 | v37.89,40.69 39.86,40.69 v43.23,44.38 48.95,44.38 55.01,50.46 55.01,57.99 55,58 | 28.65,66.38 27.73,67.31 27.73,70.13 26.2,71.66 23.85,71.66 v23.83,71.64 | v26.77,66.38 28.65,66.38 | 28.65,66.38 29.1,65.94
-VS  (via drill 0.6)
  Top 0.406: U$1.3 38.76,50.99 39.08,50.68 C25.1 | R16.1 28.89,63.57 v29.68,62.71
  Top 0.61: 43.33,34.04 C3.1 42.14,34.06 39.99,35.94 40,43 38,45 | 22.62,45.81 R8.1 23.19,45.81 24,45 v27,45 27,47 26.16,47.84 C12.2 23.67,47.85 | C25.1 39.08,46.08 38,45 | 38,45 v36.84,45 | 21.56,51.3 U$10.4 21.54,50.71 v23.68,50.71 | 23.68,49.3 C13.2 | v29.69,57.03 C16.2 C17.2 29.31,54.71 U$12.4
  Top 0.813: v23.68,50.71 23.68,49.3
  Top 1.016: U$2.P$2 43.33,34.04 | C13.2 23.67,47.85
  Bottom 0.406: v23.68,50.71 25.24,52.26 28.05,52.26 29.31,53.52 29.31,56.64 v29.69,57.03
  Bottom 0.61: v36.84,45 v27,45 | v29.68,62.71 v29.69,57.03
A6
  Top 0.61: THUMBJOYSTICK.H2 32,20 26.12,28.35 22.74,28.35 21.84,29 21.84,30.5 20.23,32.21 U$13.5/A7
  Top 0.813: U$13.5/A7
A7
  Top 0.61: U$13.6/A6 18.77,29.67 19.8,28.74 19.8,24.81 20.61,24 THUMBJOYSTICK.V2
BTN  (via drill 0.5)
  Top 0.406: THUMBJOYSTICK.B1A 16.05,36.7 13.52,34.52 v13.52,29.68
  Bottom 0.254: THUMBJOYSTICK.B1A 28.82,36.83
  Bottom 0.406: v13.52,29.68 13.52,24.19 15.65,22.05 U$13.9/A3
CARD_CS
  Bottom 0.254: DISPLAY.5 2.9,61.27 0.9,58.73 0.9,16.07 1.01,15.96 1.5,15.47 U$13.12/D9
COMP_IN
  Top 0.406: VFC.7 18.95,64.2
  Top 1.016: 18.95,64.2 R1.1
D/C
  Top 0.406: U$13.7/D4 4.89,27.13 6,28.25 6,36 4,38 4,45.7 7,48.7 7,63 6.19,63.81 DISPLAY.4 | U$13.7/D4
DGND  (via drill 0.5)
  Top 0.406: 39.04,61.6 C33.1 | MCDC01.9 43.41,68.59 43,69 v43,70 | MCDC01.7 MCDC01.8
  Top 0.61: 39.01,72.98 v39.01,72.92 | 49.03,69.33 MCDC01.8
  Top 0.813: v40.55,61.6 39.04,61.6 | R21.2 v49.03,70.25 49.03,69.33 | C39.1 39.01,72.98
  other vias: 5.85,22.91 5.81,19.69 35.35,75.37 59.64,58.94 61.64,63.94 61.64,54.94 61.64,71.94 57.64,16.94 61.64,7.94 40.64,25.94 40.64,23.94 40.64,21.94 47.46,17.31 35.69,78.79 55.73,29.49 59.64,47.94 59.64,40.94 59.64,32.94 8.17,39.78 7.34,66.88 11.84,48.77
  pour Top (rank 2): 0.5,79.5 9.25,79.5 9.25,5 0.5,5
  pour Bottom (rank 2): 0.5,79.5 9.25,79.5 9.25,5 0.5,5
  pour Top (rank 2): 0.5,44 19,44 19,38 36,38 44.55,30.5 63.5,30.5 63.5,0.5 0.5,0.5
  pour Bottom (rank 2): 0.5,44 19,44 19,38 36,38.01 44.55,30.5 63.5,30.5 63.5,0.5 0.5,0.5
  pour Bottom (rank 2): 57,79.5 57,23 63.5,23 63.5,79.5
  pour Top (rank 2): 57,79.5 63.5,79.5 63.5,23 57,23
  pour Top (rank 2): 0.5,55 9.22,54.8 15.25,48.83 15.25,41.73 0.5,41.73
  pour Bottom (rank 2): 0.5,55 9.16,54.84 15.25,48.87 15.25,41.73 0.5,41.73
  pour Bottom (rank 2): 56.75,79.5 56.75,60.75 37.02,60.75 30,68 30,78 7,78 7,79.5
  pour Top (rank 2): 57,79.5 57,60.75 37,60.75 30,68 30,78 7,78 7,79.5
  pour Top (rank 2): 7,79.5 7,78 30,78 30,68 37,60.75 56.75,60.75 56.75,79.5
  pour Top (rank 2): 8.32,79.5 8.32,78 30.04,78 30,75 36.62,75 36.62,75 37,75 37,79.5
  pour Top (rank 2): 8.32,79.5 8.32,78 30,78 30,75 36.62,75 36.62,75 37,75 37,79.5
DGND_IN
  Top 0.61: U$11.2 49.15,26.7 U$6.4
DX
  Top 0.406: R15.1 27.03,50.97 28,50 30.16,50 30.58,49.58 31,50 34,50 34.96,49.04 U$1.6
  Top 0.61: U$12.6 30.58,49.58
FOUT
  Top 0.406: U$13.8/D5 5.54,24.59 7.62,26.67 7.62,35.75 5,38.37 5,45 8.68,48.68 8.68,68.97 | R3.1 8.66,74.7 10.16,76.2 15.24,76.2 16.41,75.03 VFC.3
  Top 0.61: 8.68,68.97 R3.1
GND  (via drill 0.5)
  other vias: 15.23,68.05 43.19,53.65 46.98,47.02 55.73,39.48 55.73,37.48 55.73,35.48 55.73,33.48 55.73,41.48 53.73,42.48 51.73,42.48 37.98,39.02 26.98,39.02 49.81,54.87 41.45,39.88 41.46,36.91 55.73,31.48 49.73,42.48
  pour Top (rank 3): 0.5,0.5 63.5,0.5 63.5,79.5 0.5,79.5
  pour Bottom (rank 3): 0.5,0.5 63.5,0.5 63.5,79.5 0.5,79.5
GNDA  (via drill 0.5)
  Top 0.406: MCDC01.6 48.12,67.29 v47.33,68.08 | R21.1 46.73,71.61
  Top 0.61: v45.48,62.84 44.84,62.84 44,62 44,61.71 C34.1
  Top 0.813: v47.33,68.08 47.33,70.57 R21.1
  Top 1.016: 46.73,71.61 R22.2 | C34.1 C35.1
  other vias: 46.33,65.08
  pour Bottom (isolate 0.254): 48,72 48,60.75 41.75,60.75 41.75,64.88 45,64.88 45,72
IN3
  Top 0.406: RELAY.10 52.48,62.6 51.02,64.06 49.85,64.06 MCDC01.1
IN+INTE
  Top 0.254: 20.31,51.25 20.31,52.31 20.71,52.71 22.13,52.71 22.5,52.35 27.74,52.35 27.93,52.35 28.27,52.69 28.27,54.02 27.96,54.43 22.61,54.43 22.47,54.44 17.8,54.44 16.95,53.42 16.95,50.39 17.34,49.98 20.15,49.98 20.27,50.1 | 20.31,51.25 20.29,51.23 | 20.27,50.19 20.33,50.14 20.33,51.23 U$10.3 20.31,51.25 | 20.27,50.1 20.27,51.32 20.33,51.38 | 20.27,50.1 20.27,50.02 20.29,50
  Top 0.61: U$10.3 20.29,51.27 20.29,50 C14.2
  Top 0.813: C14.2 18.67,48.88 R10.2
IN+TIA
  Top 0.254: 33.88,58.84 53,58.84 54,58 54,53 52,51 52,49 51,48 48.99,48 48.43,48.55 48.43,53.13 49,53.71 50.66,53.71 51.55,54.53 51.55,55.36 51.54,55.36 51.53,55.36 50.87,56.12 35.86,56.12 | 35.86,56.12 35.85,56.12 | 30.6,53.88 30.59,53.88 30.59,53.07 31.18,52.49 33.58,52.49 33.57,52.48 33.94,52.86 33.94,54.42 34.74,55.22 | 35.85,56.12 35.66,56.12 34.74,55.22 | 34.74,55.22 34.72,55.19 | 35.85,56.12 35.86,56.12
  Top 0.406: 33.36,58.42 30.57,55.64 30.57,53.82
  Top 0.61: 30.6,53.83 U$12.3 | 30.59,53.88 30.59,53.83 U$12.3 | C15.2 33.36,58.42 | 30.57,53.82 U$12.3
  Top 1.016: C15.2 32.27,58.66 R18.2
IN-TIA
  Top 0.61: R14.2 | 37.97,56.95 C21.1 | 37.86,56.96 33.7,56.96 31.84,55.1 31.84,54.82 U$12.2
  Top 0.813: R27.2
  Top 1.016: C21.1 37.86,56.96 R14.2 C22.1 R30.2 43.02,57.06 C23.1 45.38,56.96 R20.2 RELAY.12 52.48,53.6 50.82,51.94 C20.1
  Top 1.27: R27.2 C20.1
INT_RDY
  Bottom 0.406: U$13.13/D10 7.16,11.89 10.16,8.89 27.94,8.89 29.21,7.62 29.21,6.52 U$3.7
  Bottom 0.61: U$13.13/D10
IPD
  Top 0.813: 45,77.44 CON.SIG_T
  Top 1.016: RELAY.7 52.49,71.74 50.48,73.75 46.25,73.75 45,75 45,77.44
LDO_OUT3V1
  Top 0.406: C37.2 37.25,70.5 36.64,70.97 35.28,70.97
  Top 0.61: 35.28,70.97 LDO1.5
  Top 1.016: C38.2 LR3.1 C39.2 C37.2
LITE
  Top 0.406: DISPLAY.10 4.09,48.54 2.54,46.99 2.54,38.1 4.76,35.88 4.76,30.8 3.46,29.7 U$13.6/D3
MISO  (via drill 0.5)
  Top 0.406: 12.5,45.01 12.5,46.5 11.95,47.02 9.45,47.02 v8.45,46.02
  Top 0.61: 12.5,45.01 U$13.1/D12/MISO
  Bottom 0.406: DISPLAY.9 6.11,51.08 8.46,48.73 8.46,47.03 v8.45,46.02
MOSI
  Bottom 0.406: DISPLAY.7 3.16,56.16 2.5,55.5 2.5,46.68 3.81,45.37 7.05,45.37 U$13.4/D11/MOSI
MOSI_I2C_ADD
  Bottom 0.406: U$13.14/D11/MOSI 7.16,9.35 12.7,3.81 26.84,3.81
  Bottom 0.61: 26.84,3.81 U$3.10
N$1
  Top 0.406: LDO1.4 35.26,68.47 35.85,67.91 36.95,67.91
  Top 0.61: 36.95,67.91 C37.1
N$2
  Top 0.406: C5.2 20.87,55.3 20.26,55.9 19.65,55.29 D1.C | U$10.6 20.27,61.16 R1.2
  Top 0.61: 20.26,55.9 U$10.6
N$4
  Top 0.61: 50.33,39.82 C4.2 | 47.89,39.84 U$4.P$1
  Top 1.016: U$11.6 52.67,38.98 51.84,39.82 50.33,39.82 | C4.2 47.89,39.84
N$5
  cutout Top (rank 2): 38.22,79.5 38.22,60.75 56.75,60.75 56.75,79.5
N$6
  Top 0.61: U$2.P$1
  Top 1.016: U$2.P$1 C26.1 50.31,32.74 51.27,31.78 U$11.4
N$7
  Top 0.406: 53.01,1.41 R13.2 | U$14.5 51.16,2.83 51.72,2.27 51.72,1.41 R23.1
  Top 1.016: R23.1 R13.2
N$8
  Top 0.406: 13.87,64.24 R2.1
  Top 0.813: C6.1 R2.1 14,64.26 14,66 13.87,66 VFC.5
N$10
  Top 0.813: VFC.2 18.95,75.72 R6.1
N$11
  Top 0.61: R4.1 17.84,68.57 17,67.73 17,66.98 VFC.6
  Top 1.016: 23.85,68.55 R4.1 23.84,68.58 24.13,68.58 24.15,68.56 C9.1 R5.2
N$12
  Top 0.813: R6.2 R7.1
N$14
  Top 0.813: R10.1 R11.2 R9.2
N$15
  Top 0.61: R8.2 21.78,43.26 19.5,45.54 R9.1
  Top 0.813: R9.1
N$17
  Top 0.406: U$14.8 R12.2
N$18
  Top 0.406: U$14.7 53.49,4.13 U$9.1
N$21
  Top 0.813: R19.2
  Top 1.016: R19.2 R18.1 | R17.2 R19.2
N$22
  Top 0.813: R17.1 24.41,58.68 R16.2
OUT_TIA  (via drill 0.6)
  Top 0.406: R15.2 26.66,53.6 C5.1 19.6,53.6 19,52 | 19,52.31 v18,53.31
  Top 0.61: U$10.2 19,52 19,52.31
  Top 0.813: R15.2
  Bottom 0.61: VFC.1 21.49,73.22 20,71.73 13,71.73 10.5,69.53 10.5,55.5 13,53.31 v18,53.31
READY  (via drill 0.5)
  Top 0.406: MCDC01.12 v41.01,66.64 | v42,2 41.18,1 24.4,1 21.59,3.81 21.59,7.62 20.32,8.89 13.97,8.89 11.43,11.43 11.43,30.45 v9.71,32.17
  Bottom 0.305: 62.72,58.36 60.59,60.42 39.48,60.42 38,62
  Bottom 0.406: 38,62 38,65 39.64,66.64 v41.01,66.64 | 62.72,58.36 63,58.08 63,13.47 56.37,6.38 56.37,3 55.17,2 v42.01,2 v42,2 | 9.68,32.21 U$13.5/D2
  Bottom 0.61: 9.68,32.21 v9.71,32.17 | U$13.5/D2
REXT
  Top 0.406: MCDC01.5 47.36,66.64 47,67 46.99,67 45.71,68.29 45.71,69.88 R22.1
S1
  Top 0.406: U$1.4 36.49,50.35 36,50.84 36,53 36.58,53.68 41.13,53.68 41.47,54.02 C22.2
  Top 0.813: R30.1 C22.2
S2
  Top 0.406: U$1.5 35.89,49.7 34.78,50.78 34.79,53.56 36.39,55.16 C21.2
  Top 0.61: 37.96,55.26 C21.2
  Top 0.813: R14.1 37.96,55.26
S3
  Top 0.406: U$1.11 44.34,50.34 45.38,51 C23.2
  Top 0.61: 45.58,55.24 C23.2
  Top 0.813: R20.1 45.58,55.24
S4
  Top 0.406: R27.1 43.38,49.68 U$1.10
  Top 0.61: C20.2
  Top 1.016: R27.1
  Top 1.27: C20.2 R27.1
SCL
  Top 0.406: U$3.6 31,2 25.94,2 24.13,3.81 24.13,7.62 21.59,10.16 15.24,10.16 13.33,12.07 13.33,24.5 15.65,27.14 U$13.7/A5 | U$13.7/A5 | U$13.7/A5
SDA
  Top 0.406: U$3.5 32,7 30.11,8.89 25.4,8.89 22.48,11.81 16.35,11.81 15,13.12 15,23.6 16.01,24.6 U$13.8/A4 | U$13.8/A4 | U$13.8/A4
SOFT_SCL  (via drill 0.5)
  Top 0.254: 53,17.48 U$7.6
  Top 0.305: R32.1 44.5,13.3 44.83,13 | 53,17.38 U$7.6 | 51.66,14 v51.68,13.98
  Top 0.406: 53,17.48 53,15.3 v51.68,13.98 | 44.83,13 48,13 49,14 51.66,14 | MCDC01.11 42.71,67.29 42,68 v41.01,68
  Bottom 0.254: 37.91,60 56.14,60 58,58
  Bottom 0.305: 58,58 58,54 | 51.63,13.99 v51.68,13.98 | 37.91,60 36,62
  Bottom 0.406: 58,54 62,50 62,30 53,21 53,15.3 v51.68,13.98 | 51.63,13.99 48.98,13.98 46,10.75 10.07,10.75 6,14.81 6,18 4.48,19.5 U$13.10/D7 | 36,62 36,65.78 38.22,68 v41.01,68
  Bottom 0.61: U$13.10/D7
SOFT_SDA  (via drill 0.5)
  Top 0.254: 51.7,17.45 U$7.7
  Top 0.305: 51.68,16.35 v50.68,15.32
  Top 0.406: v50.68,15.32 R31.1 | U$7.7 51.68,16.35 | MCDC01.10 43.06,67.94 41,70 v40.7,70
  Bottom 0.254: 36.94,59.5 55.71,59.5 57.35,57.67
  Bottom 0.305: 57.35,57.67 57.35,53.67 | 36.94,59.5 34,62.57
  Bottom 0.406: 57.35,53.67 61,50 61,30.25 51.7,20.95 51.7,16.37 v50.68,15.32 48.76,15.35 45.41,11.75 10.48,11.75 7,15.27 7,20 5.06,22.08 2.54,22.08 | 34,62.57 34,66 38,70 v40.7,70
  Bottom 0.61: 2.54,22.08 U$13.9/D6
SPI_CLK_I2C_ADD
  Bottom 0.406: U$13.15/D13 26.38,6.81
  Bottom 0.61: 26.38,6.81 U$3.9
SPI_SCK
  Bottom 0.406: DISPLAY.8 6.07,53.62 10.16,49.53 U$13.3/D13/SCK
  Bottom 0.61: U$13.3/D13/SCK
SW_A0  (via drill 0.5)
  Top 0.254: v40.24,52.34 U$1.1
  Top 0.305: U$1.1
  Bottom 0.254: 32,38 40.53,45.54 40.53,52.05 v40.24,52.34 | 20.78,14.45 20.69,14.45 | 26,15
  Bottom 0.406: 32,38 32,21.84 26,15 25.45,14.45 20.78,14.45 | 20.69,14.45 20.28,14.45 U$13.11/A1
SW_A1  (via drill 0.5)
  Top 0.305: U$1.14 v41.83,52.34
  Bottom 0.254: v41.83,52.34 41.83,51.83 41,51 41,45.01 33.27,38
  Bottom 0.406: 33.27,38 33.27,21.16 27,14 26,13 19.21,13 U$13.12/A0
SW_EN  (via drill 0.5)
  Top 0.305: 39.36,51.64 39,51.64 | 39,51.64 U$1.2 | v39.2,51.64 39,51.64
  Top 0.406: v31,25 33,28 42.94,28 44.56,29.63 48.74,29.63 49.2,28.58
  Top 0.61: U$6.6 49.2,28.58
  Bottom 0.254: v39.2,51.64 39.5,51.5 40,51 40,46 31,38
  Bottom 0.406: 31,38 v31,25 31,22.35 28.48,19.5 18.2,19.5 17.78,19.5
  Bottom 0.61: 17.78,19.5 U$13.10/A2
TFT_CS
  Top 0.254: DISPLAY.6 2.9,58.73 0.9,56.07 0.9,18.61 U$13.11/D8
V_IN_BUCK  (via drill 0.8)
  Top 0.406: U$14.3 46.22,3.48 | U$14.2 46.73,4 46.22,3.48 | 46.22,3.48 45.09,3.48 C27.2
  Top 0.813: 40.35,3.61 42.7,3.61
  Top 1.016: 40.35,3.61 v40.32,3.6 | 42.7,3.61 C30.2 C29.2 | C29.2 | C29.2 C27.2
  Bottom 0.813: 40.32,3.32 39,1.5 30.54,1.5 29.54,3 29.54,3.65 U$3.8
  Bottom 1.016: v40.32,3.6 40.32,3.32
VDD
  Top 0.406: MCDC01.14 41.34,65.34 40.44,64.44 40.44,63.27 LR4.2
  Top 0.61: 39,64.59 LR3.2
  Top 1.016: LR3.2 C33.2 40.44,63.27
VDDA
  Top 0.406: MCDC01.15 42.69,64.69 42,64 42,63.41 LR4.1 | 42.16,61.59 C34.2
  Top 1.016: LR4.1 42.16,61.59
VPD
  Top 0.254: 51.04,68.85 51.04,71.36 49.63,72.76 45.53,72.76 43.99,74.3 43.98,74.3 43.98,74.32 43.43,74.87 | 51.04,68.85 51.9,67.99 53.16,67.99 53.99,69.16 54,69.17 54,72 51.16,74.84 | 49,63 50,63 51,62 51,61.51 52.03,60.74 53.03,60.74 53.97,61.61 54,63 51.04,65.96 51.04,68.85 | 49,63 48.53,63.42 48.53,65.42 | 51.16,74.84 46.92,74.84 46.91,74.85 | 51.18,74.84 51.16,74.84 | 49.02,61.98 49.02,62.98 49,63
  Top 0.406: MCDC01.16 46.96,64.04 49.02,61.98 C35.2
VUSB5V  (via drill 0.5)
  Top 0.305: LDO1.3 33.66,69.07 33.85,69.34 33.85,70.74 33.62,70.97 LDO1.1
  Top 0.406: U$11.1
  Top 0.61: U$6.5 50.16,27.64 51.18,29 54,29 54.67,28.32 54.67,25.15 53.68,24.16 U$11.1 | U$7.8 50.41,19.19 C1.2 47.47,19.02 | v30.89,78.75 C36.2 30.9,70.98 LDO1.1 | R3.2 5.09,68.98 5.08,69
  Top 0.813: THUMBJOYSTICK.H1 | R31.2 42.81,13.4 R32.2 42.8,10.01 | 42.83,15.34 R31.2 | THUMBJOYSTICK.V1 24.43,26.54 29.46,19.42 29.46,13.94 29.46,12.97 32.42,10.01 D2.C | U$11.1 52.66,24.15 49.69,24.15 47.47,21.93 47.47,19.02 44.45,19.02 42.81,17.41 R31.2
  Top 1.016: 29.46,13.94 THUMBJOYSTICK.H1 | D2.C 42.8,10.01
  Bottom 0.61: DISPLAY.2 4.46,69 6,69 8.27,71.27 8.27,77.81 9.06,78.75 v30.89,78.75 32.44,78.75 33.5,77.5 CON.GND_B@1
  Bottom 0.813: THUMBJOYSTICK.V1 21.84,33.54 20.61,34.74 17.78,34.74 | 4.7,66 6,66 8.49,63.51 8.49,54.83 14.53,48.79 14.53,44.73 14.5,44.7 14.5,35.8 15.57,34.74 15.58,34.75 U$13.4/+5V | CON.GND_B@1
  Bottom 1.27: THUMBJOYSTICK.V1 | 4.7,66 DISPLAY.3 | U$13.4/+5V 17.78,34.74
  pour Bottom (isolate 0.406): 41.5,80 41.5,75.35 48.55,75.35 48.55,80
  pour Top: 3,70 3,65.25 6,65.25 6,70
  pour Bottom: 3,70 3,65.25 6,65.25 6,70
X_RELAY
  Top 0.406: 54.25,17.46 U$7.5 | U$7.3
  Top 0.61: U$7.5 54.22,14.83 52.95,13.56 U$7.3 | U$7.5 54.21,21.03 57.75,24.57 57.75,67.43 RELAY.6
  Top 0.813: 60.08,69.67 RELAY.6
  Top 1.016: 60.08,69.67 D5.C
Y_RELAY
  Top 0.406: U$7.1
  Top 0.61: 61.96,56.97 D6.C | 52,10 58,10 59.47,11.47 61,13 61,52 59.74,53.26 RELAY.1 | 52,10 51.29,10 50.41,10.88 U$7.1 | U$7.2 51.68,10.32 52,10
  Top 1.016: RELAY.1 61.96,56.97

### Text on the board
tPlace: CON | IC2 | IC1 | Relay | Display | IC3 | IC4 | IC5 | LX | LX | IC6 | DC/DC-Wandler | Thumb Joystick | Arduino Nano | IC7 | L1 | IC9 | Wannenbuchse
